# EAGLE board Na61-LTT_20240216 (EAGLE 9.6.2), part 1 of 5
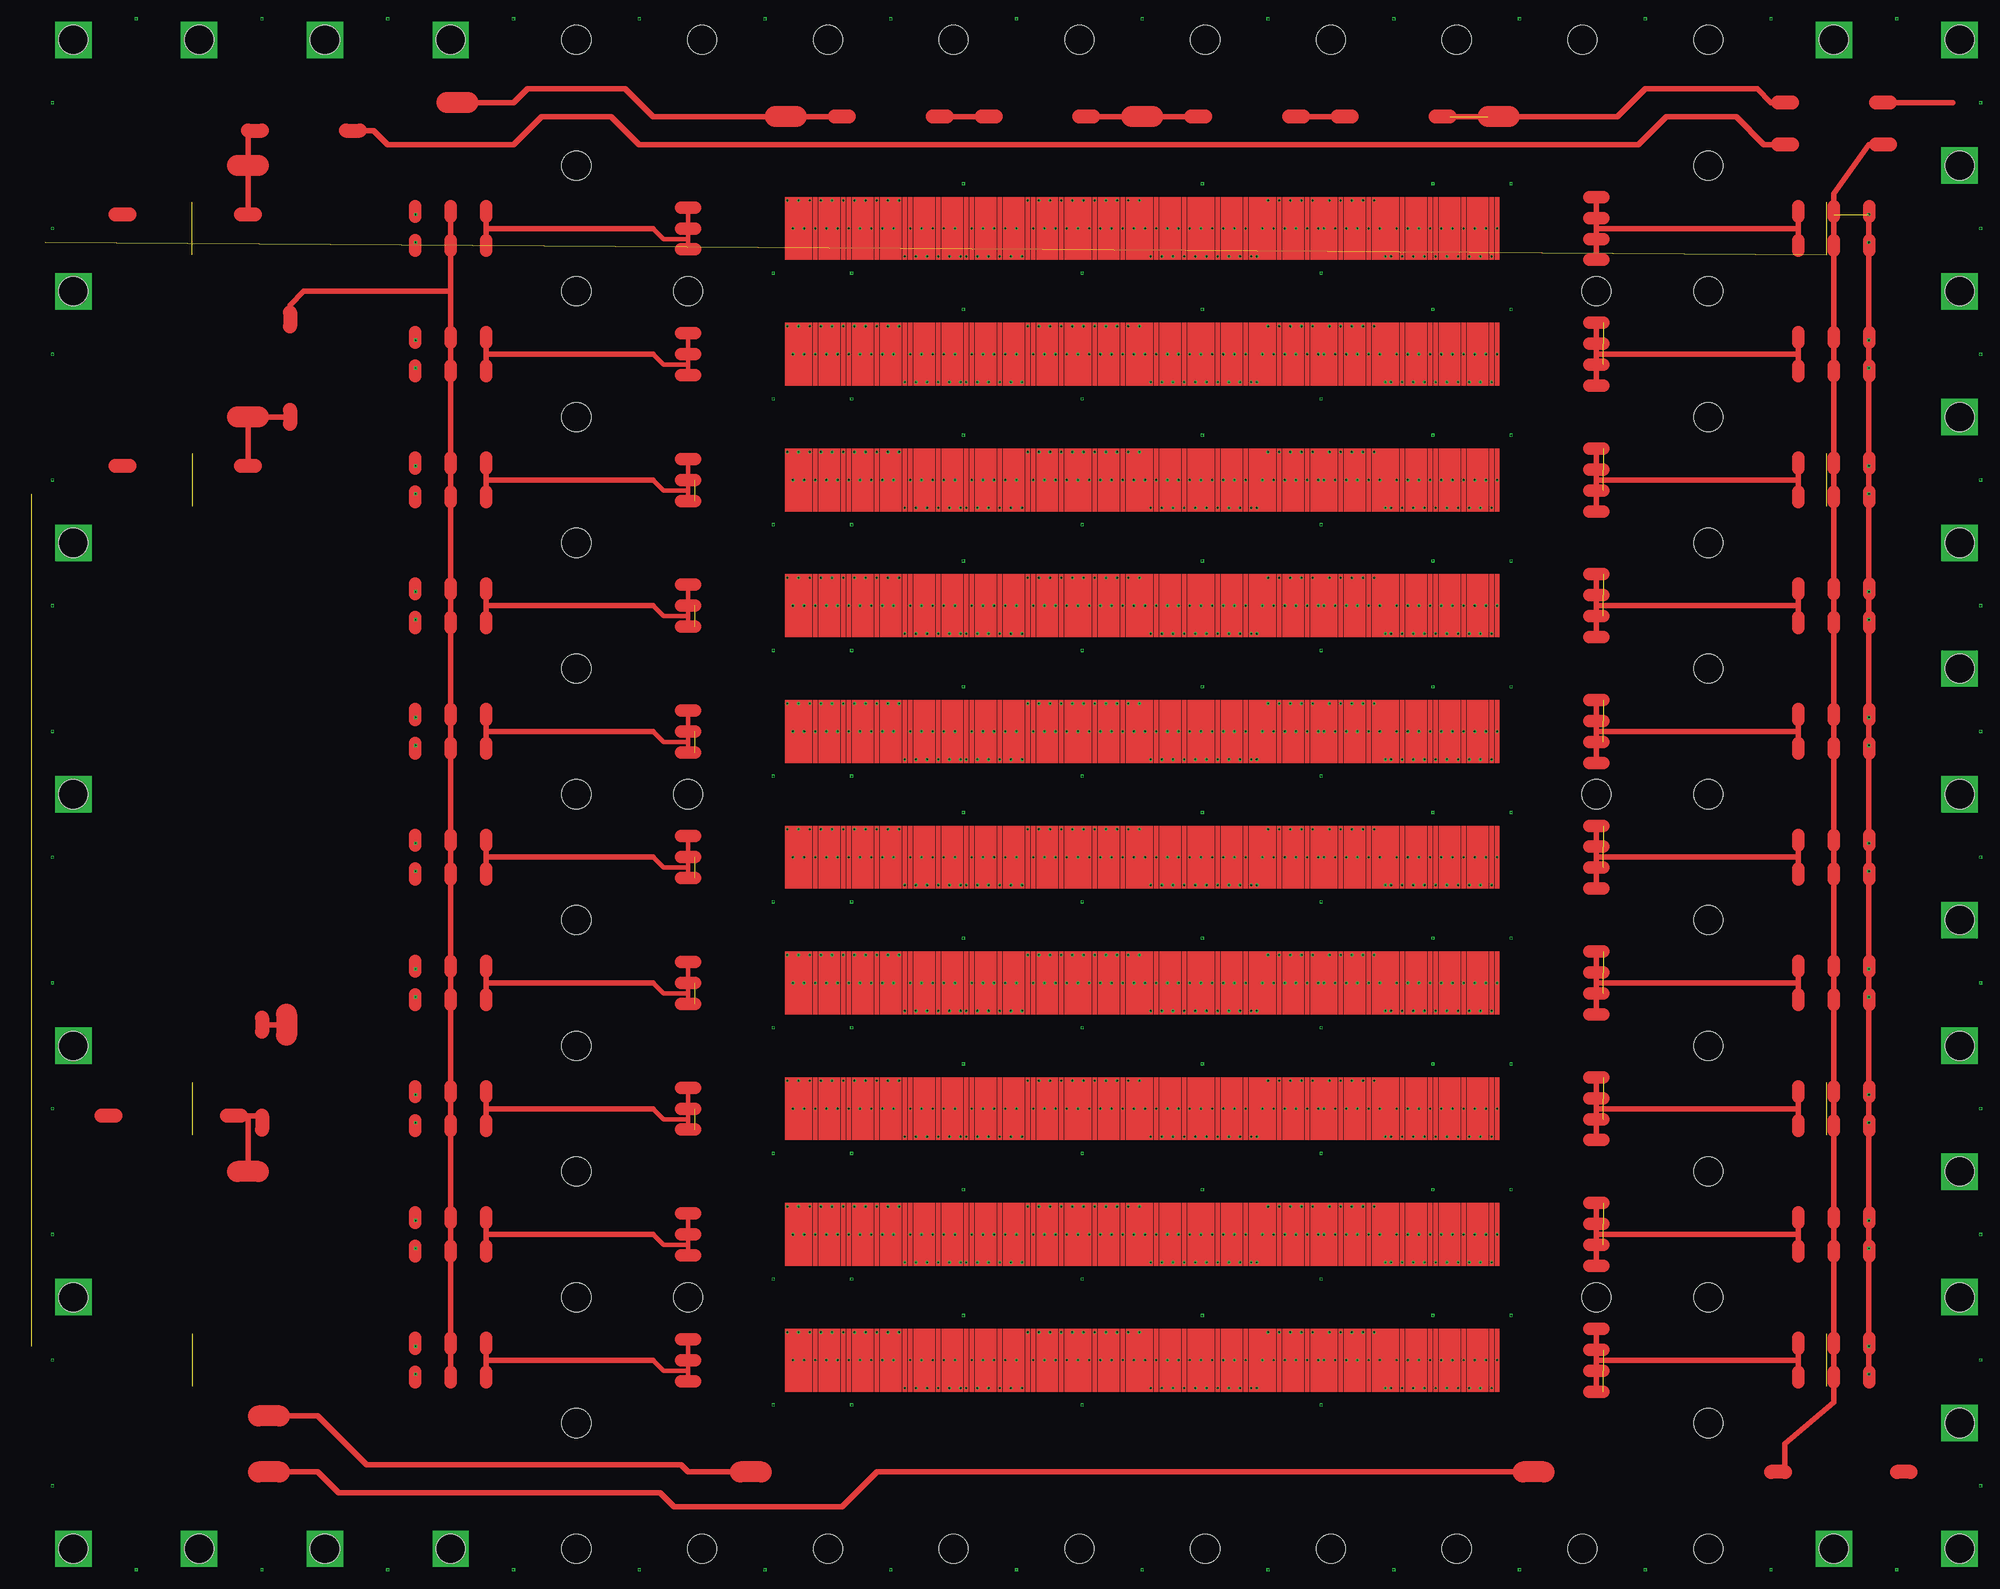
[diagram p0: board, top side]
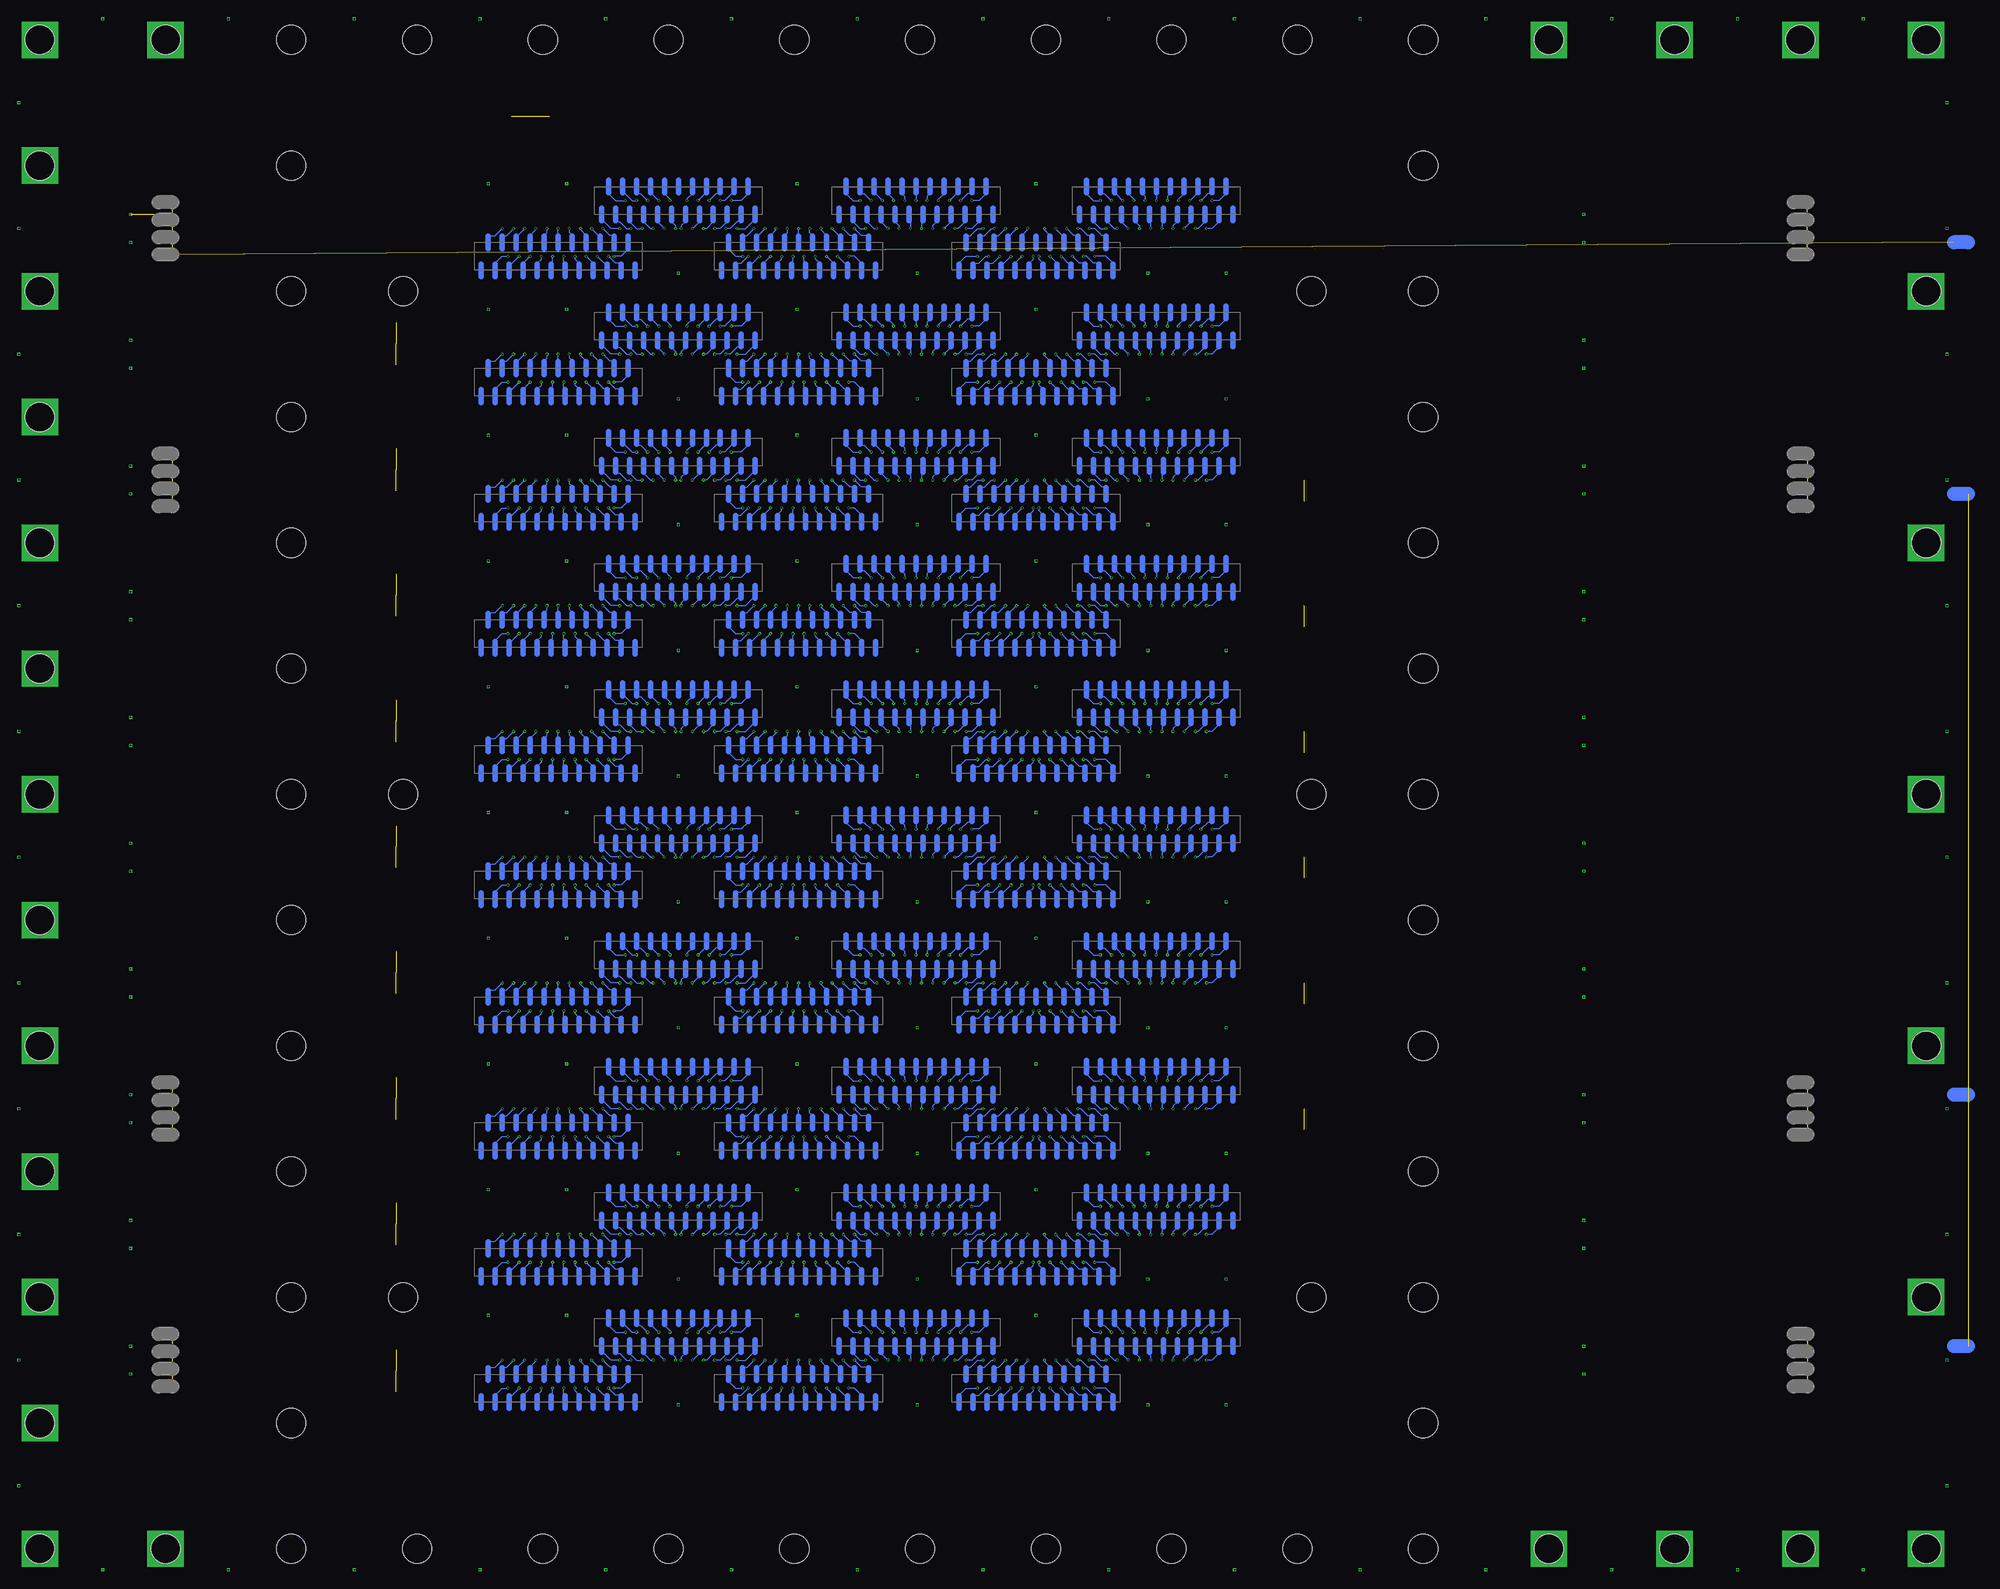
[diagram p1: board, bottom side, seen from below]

No outline drawn. Coordinates in mm, seen from the top.
Copper layers (1*16): Top 0.035mm / dielectric 1.5mm / Bottom 0.035mm
Design rules "default *": minimum track width 6mil, minimum drill 0.2mm, track to track 6mil, track to pad 6mil, pad to pad 6mil, via to via 6mil, smd to smd 6mil, copper to edge 40mil, drill to drill 6mil, minimum pad ring 8mil, minimum via ring 4mil, stop-mask expansion 4mil, vias tented up to drill 0mil, thermal gap 10mil
Holes 4.2 mm at -81,9 81,9 -81,27 -81,45 -81,63 -81,81 -81,99 -81,117 -81,135 -81,153 81,27 81,45 81,63 81,81 81,99 81,117 81,135 81,153 -81,171 81,171 81,-9 -81,-9 -65,153 65,153 -65,9 65,9 -65,81 65,81 -81,189 -63,189 -45,189 -27,189 -9,189 9,189 27,189 45,189 63,189 81,189 -81,-27 -63,-27 -45,-27 -27,-27 -9,-27 9,-27 27,-27 45,-27 63,-27 81,-27 -99,189 -117,189 -135,189 -153,189 99,189 117,189 117,171 117,153 117,135 117,117 99,-27 117,9 117,27 117,45 117,63 117,81 117,99 117,-9 117,-27 -99,-27 -117,-27 -135,-27 -153,-27 -153,9 -153,45 -153,81 -153,117 -153,153

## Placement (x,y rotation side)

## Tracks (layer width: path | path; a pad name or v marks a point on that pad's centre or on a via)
S$1
  Bottom 0.8: 11.4,-5.1 11.4,-6.9
S$2
  Bottom 0.8: 10.4,-2.9 10.4,-1.1
S$3
  Bottom 0.8: 7.4,-5.1 7.4,-6.9
S$4
  Bottom 0.8: 4.4,-2.9 4.4,-1.1
S$5
  Bottom 0.8: 1.4,-5.1 1.4,-6.9
S$6
  Bottom 0.8: 0.4,-2.9 0.4,-1.1
S$7
  Bottom 0.8: -2.6,-5.1 -2.6,-6.9
S$8
  Bottom 0.8: -1.6,-2.9 -1.6,-1.1
S$9
  Bottom 0.8: 19.4,-5.1 19.4,-6.9
S$10
  Bottom 0.8: 18.4,-2.9 18.4,-1.1
S$11
  Bottom 0.8: 15.4,-5.1 15.4,-6.9
S$12
  Bottom 0.8: 14.4,-2.9 14.4,-1.1
S$13
  Bottom 0.8: 16.4,-2.9 16.4,-1.1
S$14
  Bottom 0.8: 17.4,-5.1 17.4,-6.9
S$15
  Bottom 0.8: 13.4,-5.1 13.4,-6.9
S$16
  Bottom 0.8: 12.4,-2.9 12.4,-1.1
S$17
  Bottom 0.8: 8.4,-2.9 8.4,-1.1
S$18
  Bottom 0.8: 9.4,-5.1 9.4,-6.9
S$19
  Bottom 0.8: 5.4,-5.1 5.4,-6.9
S$20
  Bottom 0.8: 6.4,-2.9 6.4,-1.1
S$21
  Bottom 0.8: 2.4,-2.9 2.4,-1.1
S$22
  Bottom 0.8: 3.4,-5.1 3.4,-6.9
S$23
  Bottom 0.8: -0.6,-5.1 -0.6,-6.9
S$24
  Bottom 0.8: -7.4,2.9 -7.4,1.1
S$25
  Bottom 0.8: -5.4,2.9 -5.4,1.1
S$26
  Bottom 0.8: -8.4,5.1 -8.4,6.9
S$27
  Bottom 0.8: -6.4,5.1 -6.4,6.9
S$28
  Bottom 0.8: -11.4,2.9 -11.4,1.1
S$29
  Bottom 0.8: -9.4,2.9 -9.4,1.1
S$30
  Bottom 0.8: -10.4,5.1 -10.4,6.9
S$31
  Bottom 0.8: -12.4,5.1 -12.4,6.9
S$32
  Bottom 0.8: -13.4,2.9 -13.4,1.1
S$33
  Bottom 0.8: -15.4,2.9 -15.4,1.1
S$34
  Bottom 0.8: -14.4,5.1 -14.4,6.9
S$35
  Bottom 0.8: -16.4,5.1 -16.4,6.9
S$36
  Bottom 0.8: -17.4,2.9 -17.4,1.1
S$37
  Bottom 0.8: -19.4,2.9 -19.4,1.1
S$38
  Bottom 0.8: -18.4,5.1 -18.4,6.9
S$39
  Bottom 0.8: 0.6,2.9 0.6,1.1
S$40
  Bottom 0.8: 2.6,2.9 2.6,1.1
S$41
  Bottom 0.8: -0.4,5.1 -0.4,6.9
S$42
  Bottom 0.8: 1.6,5.1 1.6,6.9
S$43
  Bottom 0.8: -3.4,2.9 -3.4,1.1
S$44
  Bottom 0.8: -1.4,2.9 -1.4,1.1
S$45
  Bottom 0.8: -4.4,5.1 -4.4,6.9
S$46
  Bottom 0.8: -2.4,5.1 -2.4,6.9
S$47
  Bottom 0.8: -24.6,-5.1 -24.6,-6.9
S$48
  Bottom 0.8: -22.6,-5.1 -22.6,-6.9
S$49
  Bottom 0.8: -25.6,-2.9 -25.6,-1.1
S$50
  Bottom 0.8: -23.6,-2.9 -23.6,-1.1
S$51
  Bottom 0.8: -28.6,-5.1 -28.6,-6.9
S$52
  Bottom 0.8: -26.6,-5.1 -26.6,-6.9
S$53
  Bottom 0.8: -27.6,-2.9 -27.6,-1.1
S$54
  Bottom 0.8: -29.6,-2.9 -29.6,-1.1
S$55
  Bottom 0.8: -30.6,-5.1 -30.6,-6.9
S$56
  Bottom 0.8: -32.6,-5.1 -32.6,-6.9
S$57
  Bottom 0.8: -31.6,-2.9 -31.6,-1.1
S$58
  Bottom 0.8: -33.6,-2.9 -33.6,-1.1
S$59
  Bottom 0.8: -34.6,-5.1 -34.6,-6.9
S$60
  Bottom 0.8: -36.6,-5.1 -36.6,-6.9
S$61
  Bottom 0.8: -35.6,-2.9 -35.6,-1.1
S$62
  Bottom 0.8: -16.6,-5.1 -16.6,-6.9
S$63
  Bottom 0.8: -14.6,-5.1 -14.6,-6.9
S$64
  Bottom 0.8: -17.6,-2.9 -17.6,-1.1
S$65
  Bottom 0.8: -15.6,-2.9 -15.6,-1.1
S$66
  Bottom 0.8: -20.6,-5.1 -20.6,-6.9
S$67
  Bottom 0.8: -18.6,-5.1 -18.6,-6.9
S$68
  Bottom 0.8: -21.6,-2.9 -21.6,-1.1
S$69
  Bottom 0.8: -19.6,-2.9 -19.6,-1.1
S$70
  Bottom 0.8: 26.6,2.9 26.6,1.1
S$71
  Bottom 0.8: 28.6,2.9 28.6,1.1
S$72
  Bottom 0.8: 25.6,5.1 25.6,6.9
S$73
  Bottom 0.8: 27.6,5.1 27.6,6.9
S$74
  Bottom 0.8: 22.6,2.9 22.6,1.1
S$75
  Bottom 0.8: 24.6,2.9 24.6,1.1
S$76
  Bottom 0.8: 23.6,5.1 23.6,6.9
S$77
  Bottom 0.8: 21.6,5.1 21.6,6.9
S$78
  Bottom 0.8: 20.6,2.9 20.6,1.1
S$79
  Bottom 0.8: 18.6,2.9 18.6,1.1
S$80
  Bottom 0.8: 19.6,5.1 19.6,6.9
S$81
  Bottom 0.8: 17.6,5.1 17.6,6.9
S$82
  Bottom 0.8: 16.6,2.9 16.6,1.1
S$83
  Bottom 0.8: 14.6,2.9 14.6,1.1
S$84
  Bottom 0.8: 15.6,5.1 15.6,6.9
S$85
  Bottom 0.8: 34.6,2.9 34.6,1.1
S$86
  Bottom 0.8: 36.6,2.9 36.6,1.1
S$87
  Bottom 0.8: 33.6,5.1 33.6,6.9
S$88
  Bottom 0.8: 35.6,5.1 35.6,6.9
S$89
  Bottom 0.8: 30.6,2.9 30.6,1.1
S$90
  Bottom 0.8: 32.6,2.9 32.6,1.1
S$91
  Bottom 0.8: 29.6,5.1 29.6,6.9
S$92
  Bottom 0.8: 31.6,5.1 31.6,6.9
S$93
  Bottom 0.8: -41.8,2.9 -41.8,1.1
S$94
  Bottom 0.8: -39.8,2.9 -39.8,1.1
S$95
  Bottom 0.8: -42.8,5.1 -42.8,6.9
S$96
  Bottom 0.8: -40.8,5.1 -40.8,6.9
S$97
  Bottom 0.8: -45.8,2.9 -45.8,1.1
S$98
  Bottom 0.8: -43.8,2.9 -43.8,1.1
S$99
  Bottom 0.8: -44.8,5.1 -44.8,6.9
S$100
  Bottom 0.8: -46.8,5.1 -46.8,6.9
S$101
  Bottom 0.8: -47.8,2.9 -47.8,1.1
S$102
  Bottom 0.8: -49.8,2.9 -49.8,1.1
S$103
  Bottom 0.8: -48.8,5.1 -48.8,6.9
S$104
  Bottom 0.8: -50.8,5.1 -50.8,6.9
S$105
  Bottom 0.8: -51.8,2.9 -51.8,1.1
S$106
  Bottom 0.8: -53.8,2.9 -53.8,1.1
S$107
  Bottom 0.8: -52.8,5.1 -52.8,6.9
S$108
  Bottom 0.8: -33.8,2.9 -33.8,1.1
S$109
  Bottom 0.8: -31.8,2.9 -31.8,1.1
S$110
  Bottom 0.8: -34.8,5.1 -34.8,6.9
S$111
  Bottom 0.8: -32.8,5.1 -32.8,6.9
S$112
  Bottom 0.8: -37.8,2.9 -37.8,1.1
S$113
  Bottom 0.8: -35.8,2.9 -35.8,1.1
S$114
  Bottom 0.8: -38.8,5.1 -38.8,6.9
S$115
  Bottom 0.8: -36.8,5.1 -36.8,6.9
S$116
  Bottom 0.8: 43.8,-5.1 43.8,-6.9
S$117
  Bottom 0.8: 45.8,-5.1 45.8,-6.9
S$118
  Bottom 0.8: 42.8,-2.9 42.8,-1.1
S$119
  Bottom 0.8: 44.8,-2.9 44.8,-1.1
S$120
  Bottom 0.8: 39.8,-5.1 39.8,-6.9
S$121
  Bottom 0.8: 41.8,-5.1 41.8,-6.9
S$122
  Bottom 0.8: 40.8,-2.9 40.8,-1.1
S$123
  Bottom 0.8: 38.8,-2.9 38.8,-1.1
S$124
  Bottom 0.8: 37.8,-5.1 37.8,-6.9
S$125
  Bottom 0.8: 35.8,-5.1 35.8,-6.9
S$126
  Bottom 0.8: 36.8,-2.9 36.8,-1.1
S$127
  Bottom 0.8: 34.8,-2.9 34.8,-1.1
S$128
  Bottom 0.8: 33.8,-5.1 33.8,-6.9
S$129
  Bottom 0.8: 31.8,-5.1 31.8,-6.9
S$130
  Bottom 0.8: 32.8,-2.9 32.8,-1.1
S$131
  Bottom 0.8: 51.8,-5.1 51.8,-6.9
S$132
  Bottom 0.8: 53.8,-5.1 53.8,-6.9
S$133
  Bottom 0.8: 50.8,-2.9 50.8,-1.1
S$134
  Bottom 0.8: 52.8,-2.9 52.8,-1.1
S$135
  Bottom 0.8: 47.8,-5.1 47.8,-6.9
S$136
  Bottom 0.8: 49.8,-5.1 49.8,-6.9
S$137
  Bottom 0.8: 46.8,-2.9 46.8,-1.1
S$138
  Bottom 0.8: 48.8,-2.9 48.8,-1.1
S$139
  Top 0.61: -65,3 -65,-1.5 | -65,-1.5 -65,-3 | -65,-1.5 -68.5,-1.5 -70,0
  Top 0.813: -70,0 -93.5,0
  Top 1.8: -64,3 -65,3 -66,3 | -64,-3 -65,-3 -66,-3
S$140
  Top 1.778: -104.08,1.65 -104.08,3.17
S$141  (via drill 0.2)
  other vias: -25.6,6.4
S$142
  Top 1.778: -99,1.65 -99,3.17
S$143
  Top 1.778: -93.92,1.65 -93.92,3.17
S$144
  Top 1.778: 93.92,-3.17 93.92,-1.65
S$145
  Bottom 0.8: 9.4,12.9 9.4,11.1
S$146
  Top 1.778: 93.92,1.65 93.92,3.17
S$147
  Top 1.778: 99,-3.17 99,-1.65
S$148
  Top 1.778: 99,1.65 99,3.17
S$149
  Top 1.778: 104.08,-3.17 104.08,-1.65
S$150
  Top 1.778: 104.08,1.65 104.08,3.17
S$151  (via drill 0.2)
  other vias: -8.6,-6.4
S$152  (via drill 0.2)
  other vias: 8.6,6.4
S$153  (via drill 0.2)
  other vias: 25.6,-6.4
S$154  (via drill 0.2)
  other vias: 41.6,6.4
S$155  (via drill 0.2)
  other vias: 52.8,6.4
S$156  (via drill 0.2)
  other vias: -41.6,-6.4
S$157  (via drill 0.2)
  other vias: -52.8,-6.4
S$158
  Bottom 0.8: 11.4,12.9 11.4,11.1
S$159
  Bottom 0.8: 8.4,15.1 8.4,16.9
S$160
  Bottom 0.8: 10.4,15.1 10.4,16.9
S$161
  Bottom 0.8: 5.4,12.9 5.4,11.1
S$162  (via drill 0.2)
  other vias: -50.8,4
S$163  (via drill 0.2)
  other vias: -49.2,4
S$164  (via drill 0.2)
  other vias: -47.6,4
S$165  (via drill 0.2)
  other vias: -46,4
S$166  (via drill 0.2)
  other vias: -44.4,4
S$167  (via drill 0.2)
  other vias: -42.8,4
S$168  (via drill 0.2)
  other vias: -41.2,4
S$169  (via drill 0.2)
  other vias: -39.6,4
S$170  (via drill 0.2)
  other vias: -38,4
S$171  (via drill 0.2)
  other vias: -36.4,4
S$172  (via drill 0.2)
  other vias: -34.8,4
S$173  (via drill 0.2)
  other vias: -50,0
S$174  (via drill 0.2)
  other vias: -48.4,0
S$175  (via drill 0.2)
  other vias: -46.8,0
S$176  (via drill 0.2)
  other vias: -45.2,0
S$177  (via drill 0.2)
  other vias: -43.6,0
S$178  (via drill 0.2)
  other vias: -42,0
S$179  (via drill 0.2)
  other vias: -40.4,0
S$180  (via drill 0.2)
  other vias: -38.8,0
S$181  (via drill 0.2)
  other vias: -37.2,0
S$182  (via drill 0.2)
  other vias: -35.6,0
S$183  (via drill 0.2)
  other vias: -34,-4
S$184  (via drill 0.2)
  other vias: -32.4,-4
S$185  (via drill 0.2)
  other vias: -30.8,-4
S$186  (via drill 0.2)
  other vias: -29.2,-4
S$187  (via drill 0.2)
  other vias: -27.6,-4
S$188  (via drill 0.2)
  other vias: -33.2,0
S$189  (via drill 0.2)
  other vias: -31.6,0
S$190  (via drill 0.2)
  other vias: -30,0
S$191  (via drill 0.2)
  other vias: -28.4,0
S$192  (via drill 0.2)
  other vias: -26.8,0
S$193  (via drill 0.2)
  other vias: -26,-4
S$194  (via drill 0.2)
  other vias: -0.4,4
S$195  (via drill 0.2)
  other vias: -2,4
S$196  (via drill 0.2)
  other vias: -3.6,4
S$197  (via drill 0.2)
  other vias: -5.2,4
S$198  (via drill 0.2)
  other vias: -6.8,4
S$199  (via drill 0.2)
  other vias: -8.4,4
S$200  (via drill 0.2)
  other vias: -10,4
S$201  (via drill 0.2)
  other vias: -11.6,4
S$202  (via drill 0.2)
  other vias: -13.2,4
S$203  (via drill 0.2)
  other vias: -14.8,4
S$204  (via drill 0.2)
  other vias: -16.4,4
S$205  (via drill 0.2)
  other vias: -1.2,0
S$206  (via drill 0.2)
  other vias: -2.8,0
S$207  (via drill 0.2)
  other vias: -4.4,0
S$208  (via drill 0.2)
  other vias: -6,0
S$209  (via drill 0.2)
  other vias: -7.6,0
S$210  (via drill 0.2)
  other vias: -9.2,0
S$211  (via drill 0.2)
  other vias: -10.8,0
S$212  (via drill 0.2)
  other vias: -12.4,0
S$213  (via drill 0.2)
  other vias: -14,0
S$214  (via drill 0.2)
  other vias: -15.6,0
S$215  (via drill 0.2)
  other vias: -17.2,-4
S$216  (via drill 0.2)
  other vias: -18.8,-4
S$217  (via drill 0.2)
  other vias: -20.4,-4
S$218  (via drill 0.2)
  other vias: -22,-4
S$219  (via drill 0.2)
  other vias: -23.6,-4
S$220  (via drill 0.2)
  other vias: -18,0
S$221  (via drill 0.2)
  other vias: -19.6,0
S$222  (via drill 0.2)
  other vias: -21.2,0
S$223  (via drill 0.2)
  other vias: -22.8,0
S$224  (via drill 0.2)
  other vias: -24.4,0
S$225  (via drill 0.2)
  other vias: -25.2,-4
S$226  (via drill 0.2)
  other vias: 0.4,0
S$227  (via drill 0.2)
  other vias: 2,0
S$228  (via drill 0.2)
  other vias: 3.6,0
S$229  (via drill 0.2)
  other vias: 5.2,0
S$230  (via drill 0.2)
  other vias: 6.8,0
S$231  (via drill 0.2)
  other vias: 8.4,0
S$232  (via drill 0.2)
  other vias: 10,0
S$233  (via drill 0.2)
  other vias: 11.6,0
S$234  (via drill 0.2)
  other vias: 13.2,0
S$235  (via drill 0.2)
  other vias: 14.8,0
S$236  (via drill 0.2)
  other vias: 16.4,-4
S$237  (via drill 0.2)
  other vias: 1.2,-4
S$238  (via drill 0.2)
  other vias: 2.8,-4
S$239  (via drill 0.2)
  other vias: 4.4,-4
S$240  (via drill 0.2)
  other vias: 6,-4
S$241  (via drill 0.2)
  other vias: 7.6,-4
S$242  (via drill 0.2)
  other vias: 9.2,-4
S$243  (via drill 0.2)
  other vias: 10.8,-4
S$244  (via drill 0.2)
  other vias: 12.4,-4
S$245  (via drill 0.2)
  other vias: 14,-4
S$246  (via drill 0.2)
  other vias: 15.6,-4
S$247  (via drill 0.2)
  other vias: 17.2,0
S$248  (via drill 0.2)
  other vias: 18.8,0
S$249  (via drill 0.2)
  other vias: 20.4,0
S$250  (via drill 0.2)
  other vias: 18,4
S$251  (via drill 0.2)
  other vias: 19.6,4
S$252  (via drill 0.2)
  other vias: 21.2,4
S$253  (via drill 0.2)
  other vias: 22,0
S$254  (via drill 0.2)
  other vias: 22.8,4
S$255  (via drill 0.2)
  other vias: 23.6,0
S$256  (via drill 0.2)
  other vias: 24.4,4
S$257  (via drill 0.2)
  other vias: 25.2,0
S$258  (via drill 0.2)
  other vias: 50.8,0
S$259  (via drill 0.2)
  other vias: 49.2,0
S$260  (via drill 0.2)
  other vias: 47.6,0
S$261  (via drill 0.2)
  other vias: 46,0
S$262  (via drill 0.2)
  other vias: 44.4,0
S$263  (via drill 0.2)
  other vias: 42.8,0
S$264  (via drill 0.2)
  other vias: 41.2,0
S$265  (via drill 0.2)
  other vias: 39.6,0
S$266  (via drill 0.2)
  other vias: 38,0
S$267  (via drill 0.2)
  other vias: 36.4,0
S$268  (via drill 0.2)
  other vias: 34.8,-4
S$269  (via drill 0.2)
  other vias: 50,-4
S$270  (via drill 0.2)
  other vias: 48.4,-4
S$271  (via drill 0.2)
  other vias: 46.8,-4
S$272  (via drill 0.2)
  other vias: 45.2,-4
S$273  (via drill 0.2)
  other vias: 43.6,-4
S$274  (via drill 0.2)
  other vias: 42,-4
S$275  (via drill 0.2)
  other vias: 40.4,-4
S$276  (via drill 0.2)
  other vias: 38.8,-4
S$277  (via drill 0.2)
  other vias: 37.2,-4
S$278  (via drill 0.2)
  other vias: 35.6,-4
S$279  (via drill 0.2)
  other vias: 34,0
S$280  (via drill 0.2)
  other vias: 32.4,0
S$281  (via drill 0.2)
  other vias: 30.8,0
S$282  (via drill 0.2)
  other vias: 33.2,4
S$283  (via drill 0.2)
  other vias: 31.6,4
S$284  (via drill 0.2)
  other vias: 30,4
S$285  (via drill 0.2)
  other vias: 29.2,0
S$286  (via drill 0.2)
  other vias: 28.4,4
S$287  (via drill 0.2)
  other vias: 27.6,0
S$288  (via drill 0.2)
  other vias: 26.8,4
S$289  (via drill 0.2)
  other vias: 26,0
S$290
  Bottom 0.152: -52.8,5 -51.8,4
S$291
  Bottom 0.152: -51.8,4 -50.8,4
S$292
  Bottom 0.152: -50.8,5 -50.2,5
S$293
  Bottom 0.152: -50.2,5 -49.2,4
S$294
  Bottom 0.152: -48.8,5 -48.6,5
S$295
  Bottom 0.152: -48.6,5 -47.6,4
S$296
  Bottom 0.152: -46.8,5 -46,4.2
S$297
  Bottom 0.152: -46,4.2 -46,4
S$298
  Bottom 0.152: -44.8,5 -44.4,4.6
S$299
  Bottom 0.152: -44.4,4.6 -44.4,4
S$300
  Bottom 0.152: -42.8,5 -42.8,4
S$301
  Bottom 0.152: -40.8,5 -41.2,4.6
S$302
  Bottom 0.152: -41.2,4.6 -41.2,4
S$303
  Bottom 0.152: -38.8,5 -39.6,4.2
S$304
  Bottom 0.152: -39.6,4.2 -39.6,4
S$305
  Bottom 0.152: -36.8,5 -37,5
S$306
  Bottom 0.152: -37,5 -38,4
S$307
  Bottom 0.152: -34.8,5 -35.4,5
S$308
  Bottom 0.152: -35.4,5 -36.4,4
S$309
  Bottom 0.152: -32.8,5 -33.8,4
S$310
  Bottom 0.152: -33.8,4 -34.8,4
S$311
  Bottom 0.152: -51.8,1 -50.8,0
S$312
  Bottom 0.152: -50.8,0 -50,0
S$313
  Bottom 0.152: -49.8,1 -48.8,0
S$314
  Bottom 0.152: -48.8,0 -48.4,0
S$315
  Bottom 0.152: -47.8,1 -46.8,0
S$316
  Bottom 0.152: -45.8,1 -45.2,0.4
S$317
  Bottom 0.152: -45.2,0.4 -45.2,0
S$318
  Bottom 0.152: -43.8,1 -43.6,0.8
S$319
  Bottom 0.152: -43.6,0.8 -43.6,0
S$320
  Bottom 0.152: -41.8,1 -42,0.8
S$321
  Bottom 0.152: -42,0.8 -42,0
S$322
  Bottom 0.152: -39.8,1 -40.4,0.4
S$323
  Bottom 0.152: -40.4,0.4 -40.4,0
S$324
  Bottom 0.152: -37.8,1 -38.8,0
S$325
  Bottom 0.152: -35.8,1 -36.8,0
S$326
  Bottom 0.152: -36.8,0 -37.2,0
S$327
  Bottom 0.152: -33.8,1 -34.8,0
S$328
  Bottom 0.152: -34.8,0 -35.6,0
S$329
  Bottom 0.152: -36.6,-5 -35.6,-4
S$330
  Bottom 0.152: -35.6,-4 -34,-4
S$331
  Bottom 0.152: -34.6,-5 -33.8,-5
S$332
  Bottom 0.152: -33.8,-5 -32.8,-4
S$333
  Bottom 0.152: -32.8,-4 -32.4,-4
S$334
  Bottom 0.152: -32.6,-5 -31.8,-5
S$335
  Bottom 0.152: -31.8,-5 -30.8,-4
S$336
  Bottom 0.152: -30.6,-5 -30.2,-5
S$337
  Bottom 0.152: -30.2,-5 -29.2,-4
S$338
  Bottom 0.152: -28.6,-5 -27.6,-4
S$339
  Bottom 0.152: -26.6,-5 -26,-4.4
S$340
  Bottom 0.152: -26,-4.4 -26,-4
S$341
  Bottom 0.152: -35.6,-1 -35,-1
S$342
  Bottom 0.152: -35,-1 -34,0
S$343
  Bottom 0.152: -34,0 -33.2,0
S$344
  Bottom 0.152: -33.6,-1 -33,-1
S$345
  Bottom 0.152: -33,-1 -32,0
S$346
  Bottom 0.152: -32,0 -31.6,0
S$347
  Bottom 0.152: -31.6,-1 -31,-1
S$348
  Bottom 0.152: -31,-1 -30,0
S$349
  Bottom 0.152: -29.6,-1 -29.4,-1
S$350
  Bottom 0.152: -29.4,-1 -28.4,0
S$351
  Bottom 0.152: -27.6,-1 -26.8,-0.2
S$352
  Bottom 0.152: -26.8,-0.2 -26.8,0
S$353
  Bottom 0.152: 1.6,5 0.6,4
S$354
  Bottom 0.152: 0.6,4 -0.4,4
S$355
  Bottom 0.152: -0.4,5 -1,5
S$356
  Bottom 0.152: -1,5 -2,4
S$357
  Bottom 0.152: -2.4,5 -2.6,5
S$358
  Bottom 0.152: -2.6,5 -3.6,4
S$359
  Bottom 0.152: -4.4,5 -5.2,4.2
S$360
  Bottom 0.152: -5.2,4.2 -5.2,4
S$361
  Bottom 0.152: -6.4,5 -6.8,4.6
S$362
  Bottom 0.152: -6.8,4.6 -6.8,4
S$363
  Bottom 0.152: -8.4,5 -8.4,4
S$364
  Bottom 0.152: -10.4,5 -10,4.6
S$365
  Bottom 0.152: -10,4.6 -10,4
S$366
  Bottom 0.152: -12.4,5 -11.6,4.2
S$367
  Bottom 0.152: -11.6,4.2 -11.6,4
S$368
  Bottom 0.152: -14.4,5 -14.2,5
S$369
  Bottom 0.152: -14.2,5 -13.2,4
S$370
  Bottom 0.152: -16.4,5 -15.8,5
S$371
  Bottom 0.152: -15.8,5 -14.8,4
S$372
  Bottom 0.152: -18.4,5 -17.4,4
S$373
  Bottom 0.152: -17.4,4 -16.4,4
S$374
  Bottom 0.152: 0.6,1 -0.4,0
S$375
  Bottom 0.152: -0.4,0 -1.2,0
S$376
  Bottom 0.152: -1.4,1 -2.4,0
S$377
  Bottom 0.152: -2.4,0 -2.8,0
S$378
  Bottom 0.152: -3.4,1 -4.4,0
S$379
  Bottom 0.152: -5.4,1 -6,0.4
S$380
  Bottom 0.152: -6,0.4 -6,0
S$381
  Bottom 0.152: -7.4,1 -7.6,0.8
S$382
  Bottom 0.152: -7.6,0.8 -7.6,0
S$383
  Bottom 0.152: -9.4,1 -9.2,0.8
S$384
  Bottom 0.152: -9.2,0.8 -9.2,0
S$385
  Bottom 0.152: -11.4,1 -10.8,0.4
S$386
  Bottom 0.152: -10.8,0.4 -10.8,0
S$387
  Bottom 0.152: -13.4,1 -12.4,0
S$388
  Bottom 0.152: -15.4,1 -14.4,0
S$389
  Bottom 0.152: -14.4,0 -14,0
S$390
  Bottom 0.152: -17.4,1 -16.4,0
S$391
  Bottom 0.152: -16.4,0 -15.6,0
S$392
  Bottom 0.152: -14.6,-5 -15.6,-4
S$393
  Bottom 0.152: -15.6,-4 -17.2,-4
S$394
  Bottom 0.152: -16.6,-5 -17.4,-5
S$395
  Bottom 0.152: -17.4,-5 -18.4,-4
S$396
  Bottom 0.152: -18.4,-4 -18.8,-4
S$397
  Bottom 0.152: -18.6,-5 -19.4,-5
S$398
  Bottom 0.152: -19.4,-5 -20.4,-4
S$399
  Bottom 0.152: -20.6,-5 -21,-5
S$400
  Bottom 0.152: -21,-5 -22,-4
S$401
  Bottom 0.152: -22.6,-5 -23.6,-4
S$402
  Bottom 0.152: -24.6,-5 -25.2,-4.4
S$403
  Bottom 0.152: -25.2,-4.4 -25.2,-4
S$404
  Bottom 0.152: -15.6,-1 -16.2,-1
S$405
  Bottom 0.152: -16.2,-1 -17.2,0
S$406
  Bottom 0.152: -17.2,0 -18,0
S$407
  Bottom 0.152: -17.6,-1 -18.2,-1
S$408
  Bottom 0.152: -18.2,-1 -19.2,0
S$409
  Bottom 0.152: -19.2,0 -19.6,0
S$410
  Bottom 0.152: -19.6,-1 -20.2,-1
S$411
  Bottom 0.152: -20.2,-1 -21.2,0
S$412
  Bottom 0.152: -21.6,-1 -21.8,-1
S$413
  Bottom 0.152: -21.8,-1 -22.8,0
S$414
  Bottom 0.152: -23.6,-1 -24.4,-0.2
S$415
  Bottom 0.152: -24.4,-0.2 -24.4,0
S$416
  Bottom 0.152: 0.4,-1 1,-1
S$417
  Bottom 0.152: 1,-1 2,0
S$418
  Bottom 0.152: 2.4,-1 2.6,-1
S$419
  Bottom 0.152: 2.6,-1 3.6,0
S$420
  Bottom 0.152: 4.4,-1 5.2,-0.2
S$421
  Bottom 0.152: 5.2,-0.2 5.2,0
S$422
  Bottom 0.152: 6.4,-1 6.8,-0.6
S$423
  Bottom 0.152: 6.8,-0.6 6.8,0
S$424
  Bottom 0.152: 8.4,-1 8.4,0
S$425
  Bottom 0.152: -1.6,-1 -0.6,-1
S$426
  Bottom 0.152: -0.6,-1 0.4,0
S$427
  Bottom 0.152: -0.6,-5 0.4,-4
S$428
  Bottom 0.152: 0.4,-4 1.2,-4
S$429
  Bottom 0.152: 1.4,-5 1.8,-5
S$430
  Bottom 0.152: 1.8,-5 2.8,-4
S$431
  Bottom 0.152: 3.4,-5 4.4,-4
S$432
  Bottom 0.152: 5.4,-5 6,-4.4
S$433
  Bottom 0.152: 6,-4.4 6,-4
S$434
  Bottom 0.152: 7.4,-5 7.6,-4.8
S$435
  Bottom 0.152: 7.6,-4.8 7.6,-4
S$436
  Bottom 0.152: 9.4,-5 9.2,-4.8
S$437
  Bottom 0.152: 9.2,-4.8 9.2,-4
S$438
  Bottom 0.152: 11.4,-5 10.8,-4.4
S$439
  Bottom 0.152: 10.8,-4.4 10.8,-4
S$440
  Bottom 0.152: 13.4,-5 12.4,-4
S$441
  Bottom 0.152: 15.4,-5 15,-5
S$442
  Bottom 0.152: 15,-5 14,-4
S$443
  Bottom 0.152: 17.4,-5 16.6,-5
S$444
  Bottom 0.152: 16.6,-5 15.6,-4
S$445
  Bottom 0.152: 10.4,-1 10,-0.6
S$446
  Bottom 0.152: 10,-0.6 10,0
S$447
  Bottom 0.152: 12.4,-1 11.6,-0.2
S$448
  Bottom 0.152: 11.6,-0.2 11.6,0
S$449
  Bottom 0.152: 14.4,-1 14.2,-1
S$450
  Bottom 0.152: 14.2,-1 13.2,0
S$451
  Bottom 0.152: 16.4,-1 15.8,-1
S$452
  Bottom 0.152: 15.8,-1 14.8,0
S$453
  Bottom 0.152: 18.4,-3 17.4,-4
S$454
  Bottom 0.152: 17.4,-4 16.4,-4
S$455
  Bottom 0.152: 16.6,1 17.2,1
S$456
  Bottom 0.152: 17.2,1 18.2,0
S$457
  Bottom 0.152: 18.2,0 18.8,0
S$458
  Bottom 0.152: 18.6,1 19.6,0
S$459
  Bottom 0.152: 19.6,0 20.4,0
S$460
  Bottom 0.152: 20.6,1 21.6,0
S$461
  Bottom 0.152: 21.6,0 22,0
S$462
  Bottom 0.152: 22.6,1 23.6,0
S$463
  Bottom 0.152: 24.6,1 25.2,0.4
S$464
  Bottom 0.152: 25.2,0.4 25.2,0
S$465
  Bottom 0.152: 15.6,5 16.6,4
S$466
  Bottom 0.152: 16.6,4 18,4
S$467
  Bottom 0.152: 17.6,5 18,5
S$468
  Bottom 0.152: 18,5 19,4
S$469
  Bottom 0.152: 19,4 19.6,4
S$470
  Bottom 0.152: 19.6,5 20.2,5
S$471
  Bottom 0.152: 20.2,5 21.2,4
S$472
  Bottom 0.152: 21.6,5 21.8,5
S$473
  Bottom 0.152: 21.8,5 22.8,4
S$474
  Bottom 0.152: 23.6,5 24.4,4.2
S$475
  Bottom 0.152: 24.4,4.2 24.4,4
S$476
  Bottom 0.152: 17.2,0 16,0
S$477
  Bottom 0.152: 16,0 15,1
S$478
  Bottom 0.152: 15,1 14.6,1
S$479
  Bottom 0.152: 50.8,-1 50.2,-1
S$480
  Bottom 0.152: 50.2,-1 49.2,0
S$481
  Bottom 0.152: 48.8,-1 48.6,-1
S$482
  Bottom 0.152: 48.6,-1 47.6,0
S$483
  Bottom 0.152: 46.8,-1 46,-0.2
S$484
  Bottom 0.152: 46,-0.2 46,0
S$485
  Bottom 0.152: 44.8,-1 44.4,-0.6
S$486
  Bottom 0.152: 44.4,-0.6 44.4,0
S$487
  Bottom 0.152: 42.8,-1 42.8,0
S$488
  Bottom 0.152: 52.8,-1 51.8,-1
S$489
  Bottom 0.152: 51.8,-1 50.8,0
S$490
  Bottom 0.152: 51.8,-5 50.8,-4
S$491
  Bottom 0.152: 50.8,-4 50,-4
S$492
  Bottom 0.152: 49.8,-5 49.4,-5
S$493
  Bottom 0.152: 49.4,-5 48.4,-4
S$494
  Bottom 0.152: 47.8,-5 46.8,-4
S$495
  Bottom 0.152: 45.8,-5 45.2,-4.4
S$496
  Bottom 0.152: 45.2,-4.4 45.2,-4
S$497
  Bottom 0.152: 43.8,-5 43.6,-4.8
S$498
  Bottom 0.152: 43.6,-4.8 43.6,-4
S$499
  Bottom 0.152: 41.8,-5 42,-4.8
S$500
  Bottom 0.152: 42,-4.8 42,-4
S$501
  Bottom 0.152: 39.8,-5 40.4,-4.4
S$502
  Bottom 0.152: 40.4,-4.4 40.4,-4
S$503
  Bottom 0.152: 37.8,-5 38.8,-4
S$504
  Bottom 0.152: 35.8,-5 36.2,-5
S$505
  Bottom 0.152: 36.2,-5 37.2,-4
S$506
  Bottom 0.152: 33.8,-5 34.6,-5
S$507
  Bottom 0.152: 34.6,-5 35.6,-4
S$508
  Bottom 0.152: 40.8,-1 41.2,-0.6
S$509
  Bottom 0.152: 41.2,-0.6 41.2,0
S$510
  Bottom 0.152: 38.8,-1 39.6,-0.2
S$511
  Bottom 0.152: 39.6,-0.2 39.6,0
S$512
  Bottom 0.152: 36.8,-1 37,-1
S$513
  Bottom 0.152: 37,-1 38,0
S$514
  Bottom 0.152: 34.8,-1 35.4,-1
S$515
  Bottom 0.152: 35.4,-1 36.4,0
S$516
  Bottom 0.152: 32.8,-3 33.8,-4
S$517
  Bottom 0.152: 33.8,-4 34.8,-4
S$518
  Bottom 0.152: 34.6,1 34,1
S$519
  Bottom 0.152: 34,1 33,0
S$520
  Bottom 0.152: 33,0 32.4,0
S$521
  Bottom 0.152: 32.6,1 31.6,0
S$522
  Bottom 0.152: 31.6,0 30.8,0
S$523
  Bottom 0.152: 30.6,1 29.6,0
S$524
  Bottom 0.152: 29.6,0 29.2,0
S$525
  Bottom 0.152: 28.6,1 27.6,0
S$526
  Bottom 0.152: 26.6,1 26,0.4
S$527
  Bottom 0.152: 26,0.4 26,0
S$528
  Bottom 0.152: 35.6,5 34.6,4
S$529
  Bottom 0.152: 34.6,4 33.2,4
S$530
  Bottom 0.152: 33.6,5 33.2,5
S$531
  Bottom 0.152: 33.2,5 32.2,4
S$532
  Bottom 0.152: 32.2,4 31.6,4
S$533
  Bottom 0.152: 31.6,5 31,5
S$534
  Bottom 0.152: 31,5 30,4
S$535
  Bottom 0.152: 29.6,5 29.4,5
S$536
  Bottom 0.152: 29.4,5 28.4,4
S$537
  Bottom 0.152: 27.6,5 26.8,4.2
S$538
  Bottom 0.152: 26.8,4.2 26.8,4
S$539
  Bottom 0.152: 34,0 35.2,0
S$540
  Bottom 0.152: 35.2,0 36.2,1
S$541
  Bottom 0.152: 36.2,1 36.6,1
S$542
  Bottom 0.8: 7.4,12.9 7.4,11.1
S$543
  Bottom 0.8: 6.4,15.1 6.4,16.9
S$544
  Bottom 0.8: 4.4,15.1 4.4,16.9
S$545
  Bottom 0.8: 3.4,12.9 3.4,11.1
S$546
  Bottom 0.8: 1.4,12.9 1.4,11.1
S$547
  Bottom 0.8: 2.4,15.1 2.4,16.9
S$548
  Bottom 0.8: 0.4,15.1 0.4,16.9
S$549
  Bottom 0.8: -0.6,12.9 -0.6,11.1
S$550
  Bottom 0.8: -2.6,12.9 -2.6,11.1
S$551
  Bottom 0.8: -1.6,15.1 -1.6,16.9
S$552
  Bottom 0.8: 17.4,12.9 17.4,11.1
S$553
  Bottom 0.8: 19.4,12.9 19.4,11.1
S$554
  Bottom 0.8: 16.4,15.1 16.4,16.9
S$555
  Bottom 0.8: 18.4,15.1 18.4,16.9
S$556
  Bottom 0.8: 13.4,12.9 13.4,11.1
S$557
  Bottom 0.8: 15.4,12.9 15.4,11.1
S$558
  Bottom 0.8: 12.4,15.1 12.4,16.9
S$559
  Bottom 0.8: 14.4,15.1 14.4,16.9
S$560
  Bottom 0.8: -7.4,20.9 -7.4,19.1
S$561
  Bottom 0.8: -5.4,20.9 -5.4,19.1
S$562
  Bottom 0.8: -8.4,23.1 -8.4,24.9
S$563
  Bottom 0.8: -6.4,23.1 -6.4,24.9
S$564
  Bottom 0.8: -11.4,20.9 -11.4,19.1
S$565
  Bottom 0.8: -9.4,20.9 -9.4,19.1
S$566
  Bottom 0.8: -10.4,23.1 -10.4,24.9
S$567
  Bottom 0.8: -12.4,23.1 -12.4,24.9
S$568
  Bottom 0.8: -13.4,20.9 -13.4,19.1
S$569
  Bottom 0.8: -15.4,20.9 -15.4,19.1
S$570
  Bottom 0.8: -14.4,23.1 -14.4,24.9
S$571
  Bottom 0.8: -16.4,23.1 -16.4,24.9
S$572
  Bottom 0.8: -17.4,20.9 -17.4,19.1
S$573
  Bottom 0.8: -19.4,20.9 -19.4,19.1
S$574
  Bottom 0.8: -18.4,23.1 -18.4,24.9
S$575
  Bottom 0.8: 0.6,20.9 0.6,19.1
S$576
  Bottom 0.8: 2.6,20.9 2.6,19.1
S$577
  Bottom 0.8: -0.4,23.1 -0.4,24.9
S$578
  Bottom 0.8: 1.6,23.1 1.6,24.9
S$579
  Bottom 0.8: -3.4,20.9 -3.4,19.1
S$580
  Bottom 0.8: -1.4,20.9 -1.4,19.1
S$581
  Bottom 0.8: -4.4,23.1 -4.4,24.9
S$582
  Bottom 0.8: -2.4,23.1 -2.4,24.9
S$583
  Bottom 0.8: -24.6,12.9 -24.6,11.1
S$584
  Bottom 0.8: -22.6,12.9 -22.6,11.1
S$585
  Bottom 0.8: -25.6,15.1 -25.6,16.9
S$586
  Bottom 0.8: -23.6,15.1 -23.6,16.9
S$587
  Bottom 0.8: -28.6,12.9 -28.6,11.1
S$588
  Bottom 0.8: -26.6,12.9 -26.6,11.1
S$589
  Bottom 0.8: -27.6,15.1 -27.6,16.9
S$590
  Bottom 0.8: -29.6,15.1 -29.6,16.9
S$591
  Bottom 0.8: -30.6,12.9 -30.6,11.1
S$592
  Bottom 0.8: -32.6,12.9 -32.6,11.1
S$593
  Bottom 0.8: -31.6,15.1 -31.6,16.9
S$594
  Bottom 0.8: -33.6,15.1 -33.6,16.9
S$595
  Bottom 0.8: -34.6,12.9 -34.6,11.1
S$596
  Bottom 0.8: -36.6,12.9 -36.6,11.1
S$597
  Bottom 0.8: -35.6,15.1 -35.6,16.9
S$598
  Bottom 0.8: -16.6,12.9 -16.6,11.1
S$599
  Bottom 0.8: -14.6,12.9 -14.6,11.1
S$600
  Bottom 0.8: -17.6,15.1 -17.6,16.9
S$601
  Bottom 0.8: -15.6,15.1 -15.6,16.9
S$602
  Bottom 0.8: -20.6,12.9 -20.6,11.1
S$603
  Bottom 0.8: -18.6,12.9 -18.6,11.1
S$604
  Bottom 0.8: -21.6,15.1 -21.6,16.9
S$605
  Bottom 0.8: -19.6,15.1 -19.6,16.9
S$606
  Bottom 0.8: 26.6,20.9 26.6,19.1
S$607
  Bottom 0.8: 28.6,20.9 28.6,19.1
S$608
  Bottom 0.8: 25.6,23.1 25.6,24.9
S$609
  Bottom 0.8: 27.6,23.1 27.6,24.9
S$610
  Bottom 0.8: 22.6,20.9 22.6,19.1
S$611
  Bottom 0.8: 24.6,20.9 24.6,19.1
S$612
  Bottom 0.8: 23.6,23.1 23.6,24.9
S$613
  Bottom 0.8: 21.6,23.1 21.6,24.9
S$614
  Bottom 0.8: 20.6,20.9 20.6,19.1
S$615
  Bottom 0.8: 18.6,20.9 18.6,19.1
S$616
  Bottom 0.8: 19.6,23.1 19.6,24.9
S$617
  Bottom 0.8: 17.6,23.1 17.6,24.9
S$618
  Bottom 0.8: 16.6,20.9 16.6,19.1
S$619
  Bottom 0.8: 14.6,20.9 14.6,19.1
S$620
  Bottom 0.8: 15.6,23.1 15.6,24.9
S$621
  Bottom 0.8: 34.6,20.9 34.6,19.1
S$622
  Bottom 0.8: 36.6,20.9 36.6,19.1
S$623
  Bottom 0.8: 33.6,23.1 33.6,24.9
S$624
  Bottom 0.8: 35.6,23.1 35.6,24.9
S$625
  Bottom 0.8: 30.6,20.9 30.6,19.1
S$626
  Bottom 0.8: 32.6,20.9 32.6,19.1
S$627
  Bottom 0.8: 29.6,23.1 29.6,24.9
S$628
  Bottom 0.8: 31.6,23.1 31.6,24.9
S$629
  Bottom 0.8: -41.8,20.9 -41.8,19.1
S$630
  Bottom 0.8: -39.8,20.9 -39.8,19.1
S$631
  Bottom 0.8: -42.8,23.1 -42.8,24.9
S$632
  Bottom 0.8: -40.8,23.1 -40.8,24.9
S$633
  Bottom 0.8: -45.8,20.9 -45.8,19.1
S$634
  Bottom 0.8: -43.8,20.9 -43.8,19.1
S$635
  Bottom 0.8: -44.8,23.1 -44.8,24.9
S$636
  Bottom 0.8: -46.8,23.1 -46.8,24.9
S$637
  Bottom 0.8: -47.8,20.9 -47.8,19.1
S$638
  Bottom 0.8: -49.8,20.9 -49.8,19.1
S$639
  Bottom 0.8: -48.8,23.1 -48.8,24.9
S$640
  Bottom 0.8: -50.8,23.1 -50.8,24.9
S$641
  Bottom 0.8: -51.8,20.9 -51.8,19.1
S$642
  Bottom 0.8: -53.8,20.9 -53.8,19.1
S$643
  Bottom 0.8: -52.8,23.1 -52.8,24.9
S$644
  Bottom 0.8: -33.8,20.9 -33.8,19.1
S$645
  Bottom 0.8: -31.8,20.9 -31.8,19.1
S$646
  Bottom 0.8: -34.8,23.1 -34.8,24.9
S$647
  Bottom 0.8: -32.8,23.1 -32.8,24.9
S$648
  Bottom 0.8: -37.8,20.9 -37.8,19.1
S$649
  Bottom 0.8: -35.8,20.9 -35.8,19.1
S$650
  Bottom 0.8: -38.8,23.1 -38.8,24.9
S$651
  Bottom 0.8: -36.8,23.1 -36.8,24.9
S$652
  Bottom 0.8: 43.8,12.9 43.8,11.1
S$653
  Bottom 0.8: 45.8,12.9 45.8,11.1
S$654
  Bottom 0.8: 42.8,15.1 42.8,16.9
S$655
  Bottom 0.8: 44.8,15.1 44.8,16.9
S$656
  Bottom 0.8: 39.8,12.9 39.8,11.1
S$657
  Bottom 0.8: 41.8,12.9 41.8,11.1
S$658
  Bottom 0.8: 40.8,15.1 40.8,16.9
S$659
  Bottom 0.8: 38.8,15.1 38.8,16.9
S$660
  Bottom 0.8: 37.8,12.9 37.8,11.1
S$661
  Bottom 0.8: 35.8,12.9 35.8,11.1
S$662
  Bottom 0.8: 36.8,15.1 36.8,16.9
S$663
  Bottom 0.8: 34.8,15.1 34.8,16.9
S$664
  Bottom 0.8: 33.8,12.9 33.8,11.1
S$665
  Bottom 0.8: 31.8,12.9 31.8,11.1
S$666
  Bottom 0.8: 32.8,15.1 32.8,16.9
S$667
  Bottom 0.8: 51.8,12.9 51.8,11.1
S$668
  Bottom 0.8: 53.8,12.9 53.8,11.1
S$669
  Bottom 0.8: 50.8,15.1 50.8,16.9
S$670
  Bottom 0.8: 52.8,15.1 52.8,16.9
S$671
  Bottom 0.8: 47.8,12.9 47.8,11.1
S$672
  Bottom 0.8: 49.8,12.9 49.8,11.1
S$673
  Bottom 0.8: 46.8,15.1 46.8,16.9
S$674
  Bottom 0.8: 48.8,15.1 48.8,16.9
S$675  (via drill 0.2)
  other vias: -50.8,22
S$676  (via drill 0.2)
  other vias: -49.2,22
S$677  (via drill 0.2)
  other vias: -47.6,22
S$678  (via drill 0.2)
  other vias: -46,22
S$679  (via drill 0.2)
  other vias: -44.4,22
S$680  (via drill 0.2)
  other vias: -42.8,22
S$681  (via drill 0.2)
  other vias: -41.2,22
S$682  (via drill 0.2)
  other vias: -39.6,22
S$683  (via drill 0.2)
  other vias: -38,22
S$684  (via drill 0.2)
  other vias: -36.4,22
S$685  (via drill 0.2)
  other vias: -34.8,22
S$686  (via drill 0.2)
  other vias: -50,18
S$687  (via drill 0.2)
  other vias: -48.4,18
S$688  (via drill 0.2)
  other vias: -46.8,18
S$689  (via drill 0.2)
  other vias: -45.2,18
S$690  (via drill 0.2)
  other vias: -43.6,18
S$691  (via drill 0.2)
  other vias: -42,18
S$692  (via drill 0.2)
  other vias: -40.4,18
S$693  (via drill 0.2)
  other vias: -38.8,18
S$694  (via drill 0.2)
  other vias: -37.2,18
S$695  (via drill 0.2)
  other vias: -35.6,18
S$696  (via drill 0.2)
  other vias: -34,14
S$697  (via drill 0.2)
  other vias: -32.4,14
S$698  (via drill 0.2)
  other vias: -30.8,14
S$699  (via drill 0.2)
  other vias: -29.2,14
S$700  (via drill 0.2)
  other vias: -27.6,14
S$701  (via drill 0.2)
  other vias: -33.2,18
S$702  (via drill 0.2)
  other vias: -31.6,18
S$703  (via drill 0.2)
  other vias: -30,18
S$704  (via drill 0.2)
  other vias: -28.4,18
S$705  (via drill 0.2)
  other vias: -26.8,18
S$706  (via drill 0.2)
  other vias: -26,14
S$707  (via drill 0.2)
  other vias: -0.4,22
S$708  (via drill 0.2)
  other vias: -2,22
S$709  (via drill 0.2)
  other vias: -3.6,22
S$710  (via drill 0.2)
  other vias: -5.2,22
S$711  (via drill 0.2)
  other vias: -6.8,22
S$712  (via drill 0.2)
  other vias: -8.4,22
S$713  (via drill 0.2)
  other vias: -10,22
S$714  (via drill 0.2)
  other vias: -11.6,22
S$715  (via drill 0.2)
  other vias: -13.2,22
S$716  (via drill 0.2)
  other vias: -14.8,22
S$717  (via drill 0.2)
  other vias: -16.4,22
S$718  (via drill 0.2)
  other vias: -1.2,18
S$719  (via drill 0.2)
  other vias: -2.8,18
S$720  (via drill 0.2)
  other vias: -4.4,18
S$721  (via drill 0.2)
  other vias: -6,18
S$722  (via drill 0.2)
  other vias: -7.6,18
S$723  (via drill 0.2)
  other vias: -9.2,18
S$724  (via drill 0.2)
  other vias: -10.8,18
S$725  (via drill 0.2)
  other vias: -12.4,18
S$726  (via drill 0.2)
  other vias: -14,18
S$727  (via drill 0.2)
  other vias: -15.6,18
S$728  (via drill 0.2)
  other vias: -17.2,14
S$729  (via drill 0.2)
  other vias: -18.8,14
S$730  (via drill 0.2)
  other vias: -20.4,14
S$731  (via drill 0.2)
  other vias: -22,14
S$732  (via drill 0.2)
  other vias: -23.6,14
S$733  (via drill 0.2)
  other vias: -18,18
S$734  (via drill 0.2)
  other vias: -19.6,18
S$735  (via drill 0.2)
  other vias: -21.2,18
S$736  (via drill 0.2)
  other vias: -22.8,18
S$737  (via drill 0.2)
  other vias: -24.4,18
S$738  (via drill 0.2)
  other vias: -25.2,14
S$739  (via drill 0.2)
  other vias: 0.4,18
S$740  (via drill 0.2)
  other vias: 2,18
S$741  (via drill 0.2)
  other vias: 3.6,18
S$742  (via drill 0.2)
  other vias: 5.2,18
S$743  (via drill 0.2)
  other vias: 6.8,18
S$744  (via drill 0.2)
  other vias: 8.4,18
S$745  (via drill 0.2)
  other vias: 10,18
S$746  (via drill 0.2)
  other vias: 11.6,18
S$747  (via drill 0.2)
  other vias: 13.2,18
S$748  (via drill 0.2)
  other vias: 14.8,18
S$749  (via drill 0.2)
  other vias: 16.4,14
S$750  (via drill 0.2)
  other vias: 1.2,14
S$751  (via drill 0.2)
  other vias: 2.8,14
S$752  (via drill 0.2)
  other vias: 4.4,14
S$753  (via drill 0.2)
  other vias: 6,14
S$754  (via drill 0.2)
  other vias: 7.6,14
S$755  (via drill 0.2)
  other vias: 9.2,14
S$756  (via drill 0.2)
  other vias: 10.8,14
S$757  (via drill 0.2)
  other vias: 12.4,14
S$758  (via drill 0.2)
  other vias: 14,14
S$759  (via drill 0.2)
  other vias: 15.6,14
S$760  (via drill 0.2)
  other vias: 17.2,18
S$761  (via drill 0.2)
  other vias: 18.8,18
S$762  (via drill 0.2)
  other vias: 20.4,18
S$763  (via drill 0.2)
  other vias: 18,22
S$764  (via drill 0.2)
  other vias: 19.6,22
S$765  (via drill 0.2)
  other vias: 21.2,22
S$766  (via drill 0.2)
  other vias: 22,18
S$767  (via drill 0.2)
  other vias: 22.8,22
S$768  (via drill 0.2)
  other vias: 23.6,18
S$769  (via drill 0.2)
  other vias: 24.4,22
S$770  (via drill 0.2)
  other vias: 25.2,18
S$771  (via drill 0.2)
  other vias: 50.8,18
S$772  (via drill 0.2)
  other vias: 49.2,18
S$773  (via drill 0.2)
  other vias: 47.6,18
S$774  (via drill 0.2)
  other vias: 46,18
S$775  (via drill 0.2)
  other vias: 44.4,18
S$776  (via drill 0.2)
  other vias: 42.8,18
S$777  (via drill 0.2)
  other vias: 41.2,18
S$778  (via drill 0.2)
  other vias: 39.6,18
S$779  (via drill 0.2)
  other vias: 38,18
S$780  (via drill 0.2)
  other vias: 36.4,18
S$781  (via drill 0.2)
  other vias: 34.8,14
S$782  (via drill 0.2)
  other vias: 50,14
S$783  (via drill 0.2)
  other vias: 48.4,14
S$784  (via drill 0.2)
  other vias: 46.8,14
S$785  (via drill 0.2)
  other vias: 45.2,14
S$786  (via drill 0.2)
  other vias: 43.6,14
S$787  (via drill 0.2)
  other vias: 42,14
S$788  (via drill 0.2)
  other vias: 40.4,14
S$789  (via drill 0.2)
  other vias: 38.8,14
S$790  (via drill 0.2)
  other vias: 37.2,14
S$791  (via drill 0.2)
  other vias: 35.6,14
S$792  (via drill 0.2)
  other vias: 34,18
S$793  (via drill 0.2)
  other vias: 32.4,18
S$794  (via drill 0.2)
  other vias: 30.8,18
S$795  (via drill 0.2)
  other vias: 33.2,22
S$796  (via drill 0.2)
  other vias: 31.6,22
S$797  (via drill 0.2)
  other vias: 30,22
S$798  (via drill 0.2)
  other vias: 29.2,18
S$799  (via drill 0.2)
  other vias: 28.4,22
S$800  (via drill 0.2)
  other vias: 27.6,18
S$801  (via drill 0.2)
  other vias: 26.8,22
S$802  (via drill 0.2)
  other vias: 26,18
S$803
  Bottom 0.152: -52.8,23 -51.8,22
S$804
  Bottom 0.152: -51.8,22 -50.8,22
S$805
  Bottom 0.152: -50.8,23 -50.2,23
S$806
  Bottom 0.152: -50.2,23 -49.2,22
S$807
  Bottom 0.152: -48.8,23 -48.6,23
S$808
  Bottom 0.152: -48.6,23 -47.6,22
S$809
  Bottom 0.152: -46.8,23 -46,22.2
S$810
  Bottom 0.152: -46,22.2 -46,22
S$811
  Bottom 0.152: -44.8,23 -44.4,22.6
S$812
  Bottom 0.152: -44.4,22.6 -44.4,22
S$813
  Bottom 0.152: -42.8,23 -42.8,22
S$814
  Bottom 0.152: -40.8,23 -41.2,22.6
S$815
  Bottom 0.152: -41.2,22.6 -41.2,22
S$816
  Bottom 0.152: -38.8,23 -39.6,22.2
S$817
  Bottom 0.152: -39.6,22.2 -39.6,22
S$818
  Bottom 0.152: -36.8,23 -37,23
S$819
  Bottom 0.152: -37,23 -38,22
S$820
  Bottom 0.152: -34.8,23 -35.4,23
S$821
  Bottom 0.152: -35.4,23 -36.4,22
S$822
  Bottom 0.152: -32.8,23 -33.8,22
S$823
  Bottom 0.152: -33.8,22 -34.8,22
S$824
  Bottom 0.152: -51.8,19 -50.8,18
S$825
  Bottom 0.152: -50.8,18 -50,18
S$826
  Bottom 0.152: -49.8,19 -48.8,18
S$827
  Bottom 0.152: -48.8,18 -48.4,18
S$828
  Bottom 0.152: -47.8,19 -46.8,18
S$829
  Bottom 0.152: -45.8,19 -45.2,18.4
S$830
  Bottom 0.152: -45.2,18.4 -45.2,18
S$831
  Bottom 0.152: -43.8,19 -43.6,18.8
S$832
  Bottom 0.152: -43.6,18.8 -43.6,18
S$833
  Bottom 0.152: -41.8,19 -42,18.8
S$834
  Bottom 0.152: -42,18.8 -42,18
S$835
  Bottom 0.152: -39.8,19 -40.4,18.4
S$836
  Bottom 0.152: -40.4,18.4 -40.4,18
S$837
  Bottom 0.152: -37.8,19 -38.8,18
S$838
  Bottom 0.152: -35.8,19 -36.8,18
S$839
  Bottom 0.152: -36.8,18 -37.2,18
S$840
  Bottom 0.152: -33.8,19 -34.8,18
S$841
  Bottom 0.152: -34.8,18 -35.6,18
S$842
  Bottom 0.152: -36.6,13 -35.6,14
S$843
  Bottom 0.152: -35.6,14 -34,14
S$844
  Bottom 0.152: -34.6,13 -33.8,13
S$845
  Bottom 0.152: -33.8,13 -32.8,14
S$846
  Bottom 0.152: -32.8,14 -32.4,14
S$847
  Bottom 0.152: -32.6,13 -31.8,13
S$848
  Bottom 0.152: -31.8,13 -30.8,14
S$849
  Bottom 0.152: -30.6,13 -30.2,13
S$850
  Bottom 0.152: -30.2,13 -29.2,14
S$851
  Bottom 0.152: -28.6,13 -27.6,14
S$852
  Bottom 0.152: -26.6,13 -26,13.6
S$853
  Bottom 0.152: -26,13.6 -26,14
S$854
  Bottom 0.152: -35.6,17 -35,17
S$855
  Bottom 0.152: -35,17 -34,18
S$856
  Bottom 0.152: -34,18 -33.2,18
S$857
  Bottom 0.152: -33.6,17 -33,17
S$858
  Bottom 0.152: -33,17 -32,18
S$859
  Bottom 0.152: -32,18 -31.6,18
S$860
  Bottom 0.152: -31.6,17 -31,17
S$861
  Bottom 0.152: -31,17 -30,18
S$862
  Bottom 0.152: -29.6,17 -29.4,17
S$863
  Bottom 0.152: -29.4,17 -28.4,18
S$864
  Bottom 0.152: -27.6,17 -26.8,17.8
S$865
  Bottom 0.152: -26.8,17.8 -26.8,18
S$866
  Bottom 0.152: 1.6,23 0.6,22
S$867
  Bottom 0.152: 0.6,22 -0.4,22
S$868
  Bottom 0.152: -0.4,23 -1,23
S$869
  Bottom 0.152: -1,23 -2,22
S$870
  Bottom 0.152: -2.4,23 -2.6,23
S$871
  Bottom 0.152: -2.6,23 -3.6,22
S$872
  Bottom 0.152: -4.4,23 -5.2,22.2
S$873
  Bottom 0.152: -5.2,22.2 -5.2,22
S$874
  Bottom 0.152: -6.4,23 -6.8,22.6
S$875
  Bottom 0.152: -6.8,22.6 -6.8,22
S$876
  Bottom 0.152: -8.4,23 -8.4,22
S$877
  Bottom 0.152: -10.4,23 -10,22.6
S$878
  Bottom 0.152: -10,22.6 -10,22
S$879
  Bottom 0.152: -12.4,23 -11.6,22.2
S$880
  Bottom 0.152: -11.6,22.2 -11.6,22
S$881
  Bottom 0.152: -14.4,23 -14.2,23
S$882
  Bottom 0.152: -14.2,23 -13.2,22
S$883
  Bottom 0.152: -16.4,23 -15.8,23
S$884
  Bottom 0.152: -15.8,23 -14.8,22
S$885
  Bottom 0.152: -18.4,23 -17.4,22
S$886
  Bottom 0.152: -17.4,22 -16.4,22
S$887
  Bottom 0.152: 0.6,19 -0.4,18
S$888
  Bottom 0.152: -0.4,18 -1.2,18
S$889
  Bottom 0.152: -1.4,19 -2.4,18
S$890
  Bottom 0.152: -2.4,18 -2.8,18
S$891
  Bottom 0.152: -3.4,19 -4.4,18
S$892
  Bottom 0.152: -5.4,19 -6,18.4
S$893
  Bottom 0.152: -6,18.4 -6,18
S$894
  Bottom 0.152: -7.4,19 -7.6,18.8
S$895
  Bottom 0.152: -7.6,18.8 -7.6,18
S$896
  Bottom 0.152: -9.4,19 -9.2,18.8
S$897
  Bottom 0.152: -9.2,18.8 -9.2,18
S$898
  Bottom 0.152: -11.4,19 -10.8,18.4
S$899
  Bottom 0.152: -10.8,18.4 -10.8,18
S$900
  Bottom 0.152: -13.4,19 -12.4,18
S$901
  Bottom 0.152: -15.4,19 -14.4,18
S$902
  Bottom 0.152: -14.4,18 -14,18
S$903
  Bottom 0.152: -17.4,19 -16.4,18
S$904
  Bottom 0.152: -16.4,18 -15.6,18
S$905
  Bottom 0.152: -14.6,13 -15.6,14
S$906
  Bottom 0.152: -15.6,14 -17.2,14
S$907
  Bottom 0.152: -16.6,13 -17.4,13
S$908
  Bottom 0.152: -17.4,13 -18.4,14
S$909
  Bottom 0.152: -18.4,14 -18.8,14
S$910
  Bottom 0.152: -18.6,13 -19.4,13
S$911
  Bottom 0.152: -19.4,13 -20.4,14
S$912
  Bottom 0.152: -20.6,13 -21,13
S$913
  Bottom 0.152: -21,13 -22,14
S$914
  Bottom 0.152: -22.6,13 -23.6,14
S$915
  Bottom 0.152: -24.6,13 -25.2,13.6
S$916
  Bottom 0.152: -25.2,13.6 -25.2,14
S$917
  Bottom 0.152: -15.6,17 -16.2,17
S$918
  Bottom 0.152: -16.2,17 -17.2,18
S$919
  Bottom 0.152: -17.2,18 -18,18
S$920
  Bottom 0.152: -17.6,17 -18.2,17
S$921
  Bottom 0.152: -18.2,17 -19.2,18
S$922
  Bottom 0.152: -19.2,18 -19.6,18
S$923
  Bottom 0.152: -19.6,17 -20.2,17
S$924
  Bottom 0.152: -20.2,17 -21.2,18
S$925
  Bottom 0.152: -21.6,17 -21.8,17
S$926
  Bottom 0.152: -21.8,17 -22.8,18
S$927
  Bottom 0.152: -23.6,17 -24.4,17.8
S$928
  Bottom 0.152: -24.4,17.8 -24.4,18
S$929
  Bottom 0.152: 0.4,17 1,17
S$930
  Bottom 0.152: 1,17 2,18
S$931
  Bottom 0.152: 2.4,17 2.6,17
S$932
  Bottom 0.152: 2.6,17 3.6,18
S$933
  Bottom 0.152: 4.4,17 5.2,17.8
S$934
  Bottom 0.152: 5.2,17.8 5.2,18
S$935
  Bottom 0.152: 6.4,17 6.8,17.4
S$936
  Bottom 0.152: 6.8,17.4 6.8,18
S$937
  Bottom 0.152: 8.4,17 8.4,18
S$938
  Bottom 0.152: -1.6,17 -0.6,17
S$939
  Bottom 0.152: -0.6,17 0.4,18
S$940
  Bottom 0.152: -0.6,13 0.4,14
S$941
  Bottom 0.152: 0.4,14 1.2,14
S$942
  Bottom 0.152: 1.4,13 1.8,13
S$943
  Bottom 0.152: 1.8,13 2.8,14
S$944
  Bottom 0.152: 3.4,13 4.4,14
S$945
  Bottom 0.152: 5.4,13 6,13.6
S$946
  Bottom 0.152: 6,13.6 6,14
S$947
  Bottom 0.152: 7.4,13 7.6,13.2
S$948
  Bottom 0.152: 7.6,13.2 7.6,14
S$949
  Bottom 0.152: 9.4,13 9.2,13.2
S$950
  Bottom 0.152: 9.2,13.2 9.2,14
S$951
  Bottom 0.152: 11.4,13 10.8,13.6
S$952
  Bottom 0.152: 10.8,13.6 10.8,14
S$953
  Bottom 0.152: 13.4,13 12.4,14
S$954
  Bottom 0.152: 15.4,13 15,13
S$955
  Bottom 0.152: 15,13 14,14
S$956
  Bottom 0.152: 17.4,13 16.6,13
S$957
  Bottom 0.152: 16.6,13 15.6,14
S$958
  Bottom 0.152: 10.4,17 10,17.4
S$959
  Bottom 0.152: 10,17.4 10,18
S$960
  Bottom 0.152: 12.4,17 11.6,17.8
S$961
  Bottom 0.152: 11.6,17.8 11.6,18
S$962
  Bottom 0.152: 14.4,17 14.2,17
S$963
  Bottom 0.152: 14.2,17 13.2,18
S$964
  Bottom 0.152: 16.4,17 15.8,17
S$965
  Bottom 0.152: 15.8,17 14.8,18
S$966
  Bottom 0.152: 18.4,15 17.4,14
S$967
  Bottom 0.152: 17.4,14 16.4,14
S$968
  Bottom 0.152: 16.6,19 17.2,19
S$969
  Bottom 0.152: 17.2,19 18.2,18
S$970
  Bottom 0.152: 18.2,18 18.8,18
S$971
  Bottom 0.152: 18.6,19 19.6,18
S$972
  Bottom 0.152: 19.6,18 20.4,18
S$973
  Bottom 0.152: 20.6,19 21.6,18
S$974
  Bottom 0.152: 21.6,18 22,18
S$975
  Bottom 0.152: 22.6,19 23.6,18
S$976
  Bottom 0.152: 24.6,19 25.2,18.4
S$977
  Bottom 0.152: 25.2,18.4 25.2,18
S$978
  Bottom 0.152: 15.6,23 16.6,22
S$979
  Bottom 0.152: 16.6,22 18,22
S$980
  Bottom 0.152: 17.6,23 18,23
S$981
  Bottom 0.152: 18,23 19,22
S$982
  Bottom 0.152: 19,22 19.6,22
S$983
  Bottom 0.152: 19.6,23 20.2,23
S$984
  Bottom 0.152: 20.2,23 21.2,22
S$985
  Bottom 0.152: 21.6,23 21.8,23
S$986
  Bottom 0.152: 21.8,23 22.8,22
S$987
  Bottom 0.152: 23.6,23 24.4,22.2
S$988
  Bottom 0.152: 24.4,22.2 24.4,22
S$989
  Bottom 0.152: 17.2,18 16,18
S$990
  Bottom 0.152: 16,18 15,19
S$991
  Top 1.778: -104.08,-3.17 -104.08,-1.65
S$992
  Top 1.778: -99,-3.17 -99,-1.65
S$993
  Top 1.778: -93.92,-3.17 -93.92,-1.65
S$994
  Bottom 0.152: 15,19 14.6,19
S$995
  Bottom 0.152: 50.8,17 50.2,17
S$996
  Bottom 0.152: 50.2,17 49.2,18
S$997
  Bottom 0.152: 48.8,17 48.6,17
S$998
  Bottom 0.152: 48.6,17 47.6,18
S$999
  Bottom 0.152: 46.8,17 46,17.8
S$1000
  Bottom 0.152: 46,17.8 46,18
S$1001
  Bottom 0.152: 44.8,17 44.4,17.4
S$1002
  Bottom 0.152: 44.4,17.4 44.4,18
S$1003
  Bottom 0.152: 42.8,17 42.8,18
S$1004
  Bottom 0.152: 52.8,17 51.8,17
S$1005
  Bottom 0.152: 51.8,17 50.8,18
S$1006
  Bottom 0.152: 51.8,13 50.8,14
S$1007
  Bottom 0.152: 50.8,14 50,14
S$1008
  Bottom 0.152: 49.8,13 49.4,13
S$1009
  Bottom 0.152: 49.4,13 48.4,14
S$1010
  Bottom 0.152: 47.8,13 46.8,14
S$1011
  Bottom 0.152: 45.8,13 45.2,13.6
S$1012
  Bottom 0.152: 45.2,13.6 45.2,14
S$1013
  Bottom 0.152: 43.8,13 43.6,13.2
S$1014
  Bottom 0.152: 43.6,13.2 43.6,14
S$1015
  Bottom 0.152: 41.8,13 42,13.2
S$1016
  Bottom 0.152: 42,13.2 42,14
S$1017
  Bottom 0.152: 39.8,13 40.4,13.6
S$1018
  Bottom 0.152: 40.4,13.6 40.4,14
S$1019
  Bottom 0.152: 37.8,13 38.8,14
S$1020
  Bottom 0.152: 35.8,13 36.2,13
S$1021
  Bottom 0.152: 36.2,13 37.2,14
S$1022
  Bottom 0.152: 33.8,13 34.6,13
S$1023
  Bottom 0.152: 34.6,13 35.6,14
S$1024
  Bottom 0.152: 40.8,17 41.2,17.4
S$1025
  Bottom 0.152: 41.2,17.4 41.2,18
S$1026
  Bottom 0.152: 38.8,17 39.6,17.8
S$1027
  Bottom 0.152: 39.6,17.8 39.6,18
S$1028
  Bottom 0.152: 36.8,17 37,17
S$1029
  Bottom 0.152: 37,17 38,18
S$1030
  Bottom 0.152: 34.8,17 35.4,17
S$1031
  Bottom 0.152: 35.4,17 36.4,18
S$1032
  Bottom 0.152: 32.8,15 33.8,14
S$1033
  Bottom 0.152: 33.8,14 34.8,14
S$1034
  Bottom 0.152: 34.6,19 34,19
S$1035
  Bottom 0.152: 34,19 33,18
S$1036
  Bottom 0.152: 33,18 32.4,18
S$1037
  Bottom 0.152: 32.6,19 31.6,18
S$1038
  Bottom 0.152: 31.6,18 30.8,18
S$1039
  Bottom 0.152: 30.6,19 29.6,18
S$1040
  Bottom 0.152: 29.6,18 29.2,18
S$1041
  Bottom 0.152: 28.6,19 27.6,18
S$1042
  Bottom 0.152: 26.6,19 26,18.4
S$1043
  Bottom 0.152: 26,18.4 26,18
S$1044
  Bottom 0.152: 35.6,23 34.6,22
S$1045
  Bottom 0.152: 34.6,22 33.2,22
S$1046
  Bottom 0.152: 33.6,23 33.2,23
S$1047
  Bottom 0.152: 33.2,23 32.2,22
S$1048
  Bottom 0.152: 32.2,22 31.6,22
S$1049
  Bottom 0.152: 31.6,23 31,23
S$1050
  Bottom 0.152: 31,23 30,22
S$1051
  Bottom 0.152: 29.6,23 29.4,23
S$1052
  Bottom 0.152: 29.4,23 28.4,22
S$1053
  Bottom 0.152: 27.6,23 26.8,22.2
S$1054
  Bottom 0.152: 26.8,22.2 26.8,22
S$1055
  Bottom 0.152: 34,18 35.2,18
S$1056
  Bottom 0.152: 35.2,18 36.2,19
S$1057
  Bottom 0.152: 36.2,19 36.6,19
S$1058  (2 unrouted)
  Top 0.813: 65,22.5 65,13.5
  Top 1.8: 66,19.5 64,19.5 | 66,22.5 65,22.5 64,22.5 | 66,16.5 64,16.5 | 66,13.5 65,13.5 64,13.5
S$1059
  Top 1.778: -104.08,14.82 -104.08,16.35
S$1060
  Top 1.778: -104.08,19.65 -104.08,21.18
S$1061
  Top 1.778: -99,14.82 -99,16.35
S$1062
  Top 1.778: -99,19.65 -99,21.18
S$1063
  Top 1.778: -93.92,14.82 -93.92,16.35
S$1064
  Top 1.778: -93.92,19.65 -93.92,21.18
S$1065
  Top 1.778: 93.92,14.82 93.92,16.35
S$1066
  Top 1.778: 93.92,19.65 93.92,21.18
S$1067
  Top 1.778: 99,14.82 99,16.35
S$1068
  Top 1.778: 99,19.65 99,21.18
S$1069
  Top 1.778: 104.08,14.82 104.08,16.35
S$1070
  Top 1.778: 104.08,19.65 104.08,21.18
S$1071  (via drill 0.2)
  other vias: -25.6,24.4
S$1072  (via drill 0.2)
  other vias: -8.6,11.6
S$1073  (via drill 0.2)
  other vias: 8.6,24.4
S$1074  (via drill 0.2)
  other vias: 25.6,11.6
S$1075  (via drill 0.2)
  other vias: 41.6,24.4
S$1076  (via drill 0.2)
  other vias: 52.8,24.4
S$1077  (via drill 0.2)
  other vias: -41.6,11.6
S$1078  (via drill 0.2)
  other vias: -52.8,11.6
S$1079
  Bottom 0.8: 9.4,30.9 9.4,29.1
S$1080
  Bottom 0.8: 11.4,30.9 11.4,29.1
S$1081
  Bottom 0.8: 8.4,33.1 8.4,34.9
S$1082
  Bottom 0.8: 10.4,33.1 10.4,34.9
S$1083
  Bottom 0.8: 5.4,30.9 5.4,29.1
S$1084
  Bottom 0.8: 7.4,30.9 7.4,29.1
S$1085
  Bottom 0.8: 6.4,33.1 6.4,34.9
S$1086
  Bottom 0.8: 4.4,33.1 4.4,34.9
S$1087
  Bottom 0.8: 3.4,30.9 3.4,29.1
S$1088
  Bottom 0.8: 1.4,30.9 1.4,29.1
S$1089
  Bottom 0.8: 2.4,33.1 2.4,34.9
S$1090
  Bottom 0.8: 0.4,33.1 0.4,34.9
S$1091
  Bottom 0.8: -0.6,30.9 -0.6,29.1
S$1092
  Bottom 0.8: -2.6,30.9 -2.6,29.1
S$1093
  Bottom 0.8: -1.6,33.1 -1.6,34.9
S$1094
  Bottom 0.8: 17.4,30.9 17.4,29.1
S$1095
  Bottom 0.8: 19.4,30.9 19.4,29.1
S$1096
  Bottom 0.8: 16.4,33.1 16.4,34.9
S$1097
  Bottom 0.8: 18.4,33.1 18.4,34.9
S$1098
  Bottom 0.8: 13.4,30.9 13.4,29.1
S$1099
  Bottom 0.8: 15.4,30.9 15.4,29.1
S$1100
  Bottom 0.8: 12.4,33.1 12.4,34.9
S$1101
  Bottom 0.8: 14.4,33.1 14.4,34.9
S$1102
  Bottom 0.8: -7.4,38.9 -7.4,37.1
S$1103
  Bottom 0.8: -5.4,38.9 -5.4,37.1
S$1104
  Bottom 0.8: -8.4,41.1 -8.4,42.9
S$1105
  Bottom 0.8: -6.4,41.1 -6.4,42.9
S$1106
  Bottom 0.8: -11.4,38.9 -11.4,37.1
S$1107
  Bottom 0.8: -9.4,38.9 -9.4,37.1
S$1108
  Bottom 0.8: -10.4,41.1 -10.4,42.9
S$1109
  Bottom 0.8: -12.4,41.1 -12.4,42.9
S$1110
  Bottom 0.8: -13.4,38.9 -13.4,37.1
S$1111
  Bottom 0.8: -15.4,38.9 -15.4,37.1
S$1112
  Bottom 0.8: -14.4,41.1 -14.4,42.9
S$1113
  Bottom 0.8: -16.4,41.1 -16.4,42.9
S$1114
  Bottom 0.8: -17.4,38.9 -17.4,37.1
S$1115
  Bottom 0.8: -19.4,38.9 -19.4,37.1
S$1116
  Bottom 0.8: -18.4,41.1 -18.4,42.9
S$1117
  Bottom 0.8: 0.6,38.9 0.6,37.1
S$1118
  Bottom 0.8: 2.6,38.9 2.6,37.1
S$1119
  Bottom 0.8: -0.4,41.1 -0.4,42.9
S$1120
  Bottom 0.8: 1.6,41.1 1.6,42.9
S$1121
  Bottom 0.8: -3.4,38.9 -3.4,37.1
S$1122
  Bottom 0.8: -1.4,38.9 -1.4,37.1
S$1123
  Bottom 0.8: -4.4,41.1 -4.4,42.9
S$1124
  Bottom 0.8: -2.4,41.1 -2.4,42.9
S$1125
  Bottom 0.8: -24.6,30.9 -24.6,29.1
S$1126
  Bottom 0.8: -22.6,30.9 -22.6,29.1
S$1127
  Bottom 0.8: -25.6,33.1 -25.6,34.9
S$1128
  Bottom 0.8: -23.6,33.1 -23.6,34.9
S$1129
  Bottom 0.8: -28.6,30.9 -28.6,29.1
S$1130
  Bottom 0.8: -26.6,30.9 -26.6,29.1
S$1131
  Bottom 0.8: -27.6,33.1 -27.6,34.9
S$1132
  Bottom 0.8: -29.6,33.1 -29.6,34.9
S$1133
  Bottom 0.8: -30.6,30.9 -30.6,29.1
S$1134
  Bottom 0.8: -32.6,30.9 -32.6,29.1
S$1135
  Bottom 0.8: -31.6,33.1 -31.6,34.9
S$1136
  Bottom 0.8: -33.6,33.1 -33.6,34.9
S$1137
  Bottom 0.8: -34.6,30.9 -34.6,29.1
S$1138
  Bottom 0.8: -36.6,30.9 -36.6,29.1
S$1139
  Bottom 0.8: -35.6,33.1 -35.6,34.9
S$1140
  Bottom 0.8: -16.6,30.9 -16.6,29.1
S$1141
  Bottom 0.8: -14.6,30.9 -14.6,29.1
S$1142
  Bottom 0.8: -17.6,33.1 -17.6,34.9
S$1143
  Bottom 0.8: -15.6,33.1 -15.6,34.9
S$1144
  Bottom 0.8: -20.6,30.9 -20.6,29.1
S$1145
  Bottom 0.8: -18.6,30.9 -18.6,29.1
S$1146
  Bottom 0.8: -21.6,33.1 -21.6,34.9
S$1147
  Bottom 0.8: -19.6,33.1 -19.6,34.9
S$1148
  Bottom 0.8: 26.6,38.9 26.6,37.1
S$1149
  Bottom 0.8: 28.6,38.9 28.6,37.1
S$1150
  Bottom 0.8: 25.6,41.1 25.6,42.9
S$1151
  Bottom 0.8: 27.6,41.1 27.6,42.9
S$1152
  Bottom 0.8: 22.6,38.9 22.6,37.1
S$1153
  Bottom 0.8: 24.6,38.9 24.6,37.1
S$1154
  Bottom 0.8: 23.6,41.1 23.6,42.9
S$1155
  Bottom 0.8: 21.6,41.1 21.6,42.9
S$1156
  Bottom 0.8: 20.6,38.9 20.6,37.1
S$1157
  Bottom 0.8: 18.6,38.9 18.6,37.1
S$1158
  Bottom 0.8: 19.6,41.1 19.6,42.9
S$1159
  Bottom 0.8: 17.6,41.1 17.6,42.9
S$1160
  Bottom 0.8: 16.6,38.9 16.6,37.1
S$1161
  Bottom 0.8: 14.6,38.9 14.6,37.1
S$1162
  Bottom 0.8: 15.6,41.1 15.6,42.9
S$1163
  Bottom 0.8: 34.6,38.9 34.6,37.1
S$1164
  Bottom 0.8: 36.6,38.9 36.6,37.1
S$1165
  Bottom 0.8: 33.6,41.1 33.6,42.9
S$1166
  Bottom 0.8: 35.6,41.1 35.6,42.9
S$1167
  Bottom 0.8: 30.6,38.9 30.6,37.1
S$1168
  Bottom 0.8: 32.6,38.9 32.6,37.1
S$1169
  Bottom 0.8: 29.6,41.1 29.6,42.9
S$1170
  Bottom 0.8: 31.6,41.1 31.6,42.9
S$1171
  Bottom 0.8: -41.8,38.9 -41.8,37.1
S$1172
  Bottom 0.8: -39.8,38.9 -39.8,37.1
S$1173
  Bottom 0.8: -42.8,41.1 -42.8,42.9
S$1174
  Bottom 0.8: -40.8,41.1 -40.8,42.9
S$1175
  Bottom 0.8: -45.8,38.9 -45.8,37.1
S$1176
  Bottom 0.8: -43.8,38.9 -43.8,37.1
S$1177
  Bottom 0.8: -44.8,41.1 -44.8,42.9
S$1178
  Bottom 0.8: -46.8,41.1 -46.8,42.9
S$1179
  Bottom 0.8: -47.8,38.9 -47.8,37.1
S$1180
  Bottom 0.8: -49.8,38.9 -49.8,37.1
S$1181
  Bottom 0.8: -48.8,41.1 -48.8,42.9
S$1182
  Bottom 0.8: -50.8,41.1 -50.8,42.9
S$1183
  Bottom 0.8: -51.8,38.9 -51.8,37.1
S$1184
  Bottom 0.8: -53.8,38.9 -53.8,37.1
S$1185
  Bottom 0.8: -52.8,41.1 -52.8,42.9
S$1186
  Bottom 0.8: -33.8,38.9 -33.8,37.1
S$1187
  Bottom 0.8: -31.8,38.9 -31.8,37.1
S$1188
  Bottom 0.8: -34.8,41.1 -34.8,42.9
S$1189
  Bottom 0.8: -32.8,41.1 -32.8,42.9
S$1190
  Bottom 0.8: -37.8,38.9 -37.8,37.1
S$1191
  Bottom 0.8: -35.8,38.9 -35.8,37.1
S$1192
  Bottom 0.8: -38.8,41.1 -38.8,42.9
